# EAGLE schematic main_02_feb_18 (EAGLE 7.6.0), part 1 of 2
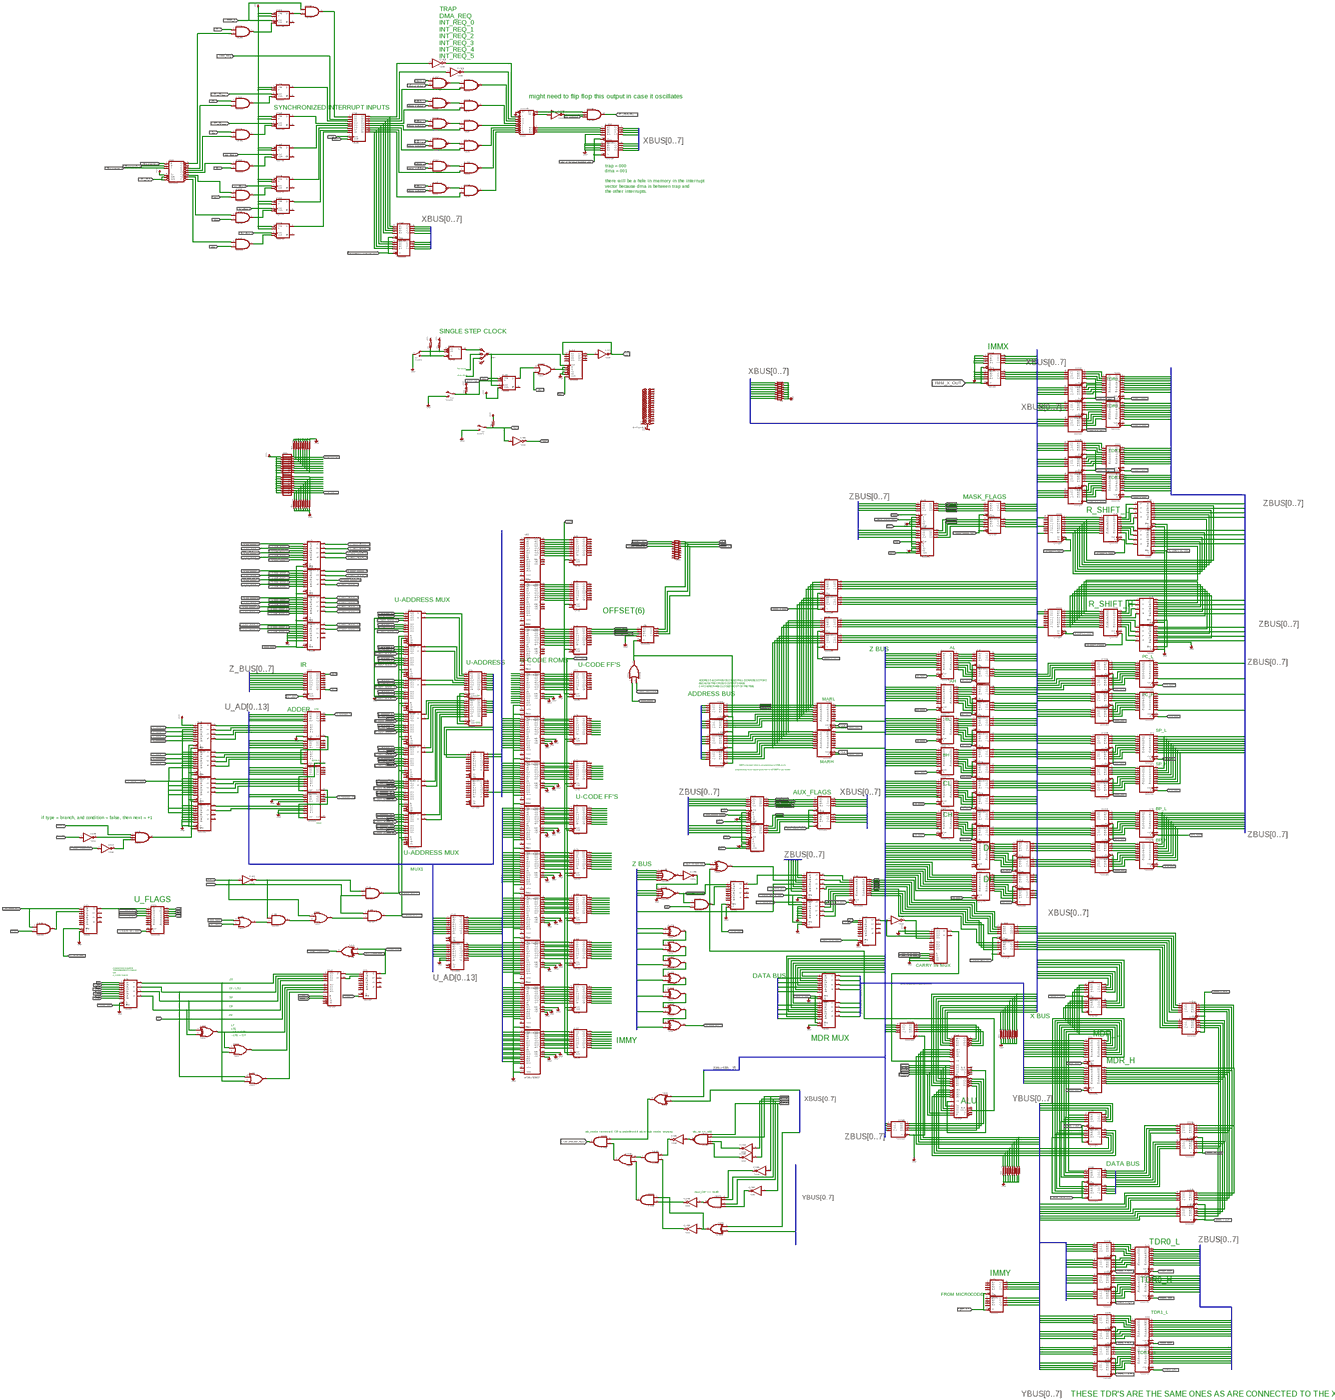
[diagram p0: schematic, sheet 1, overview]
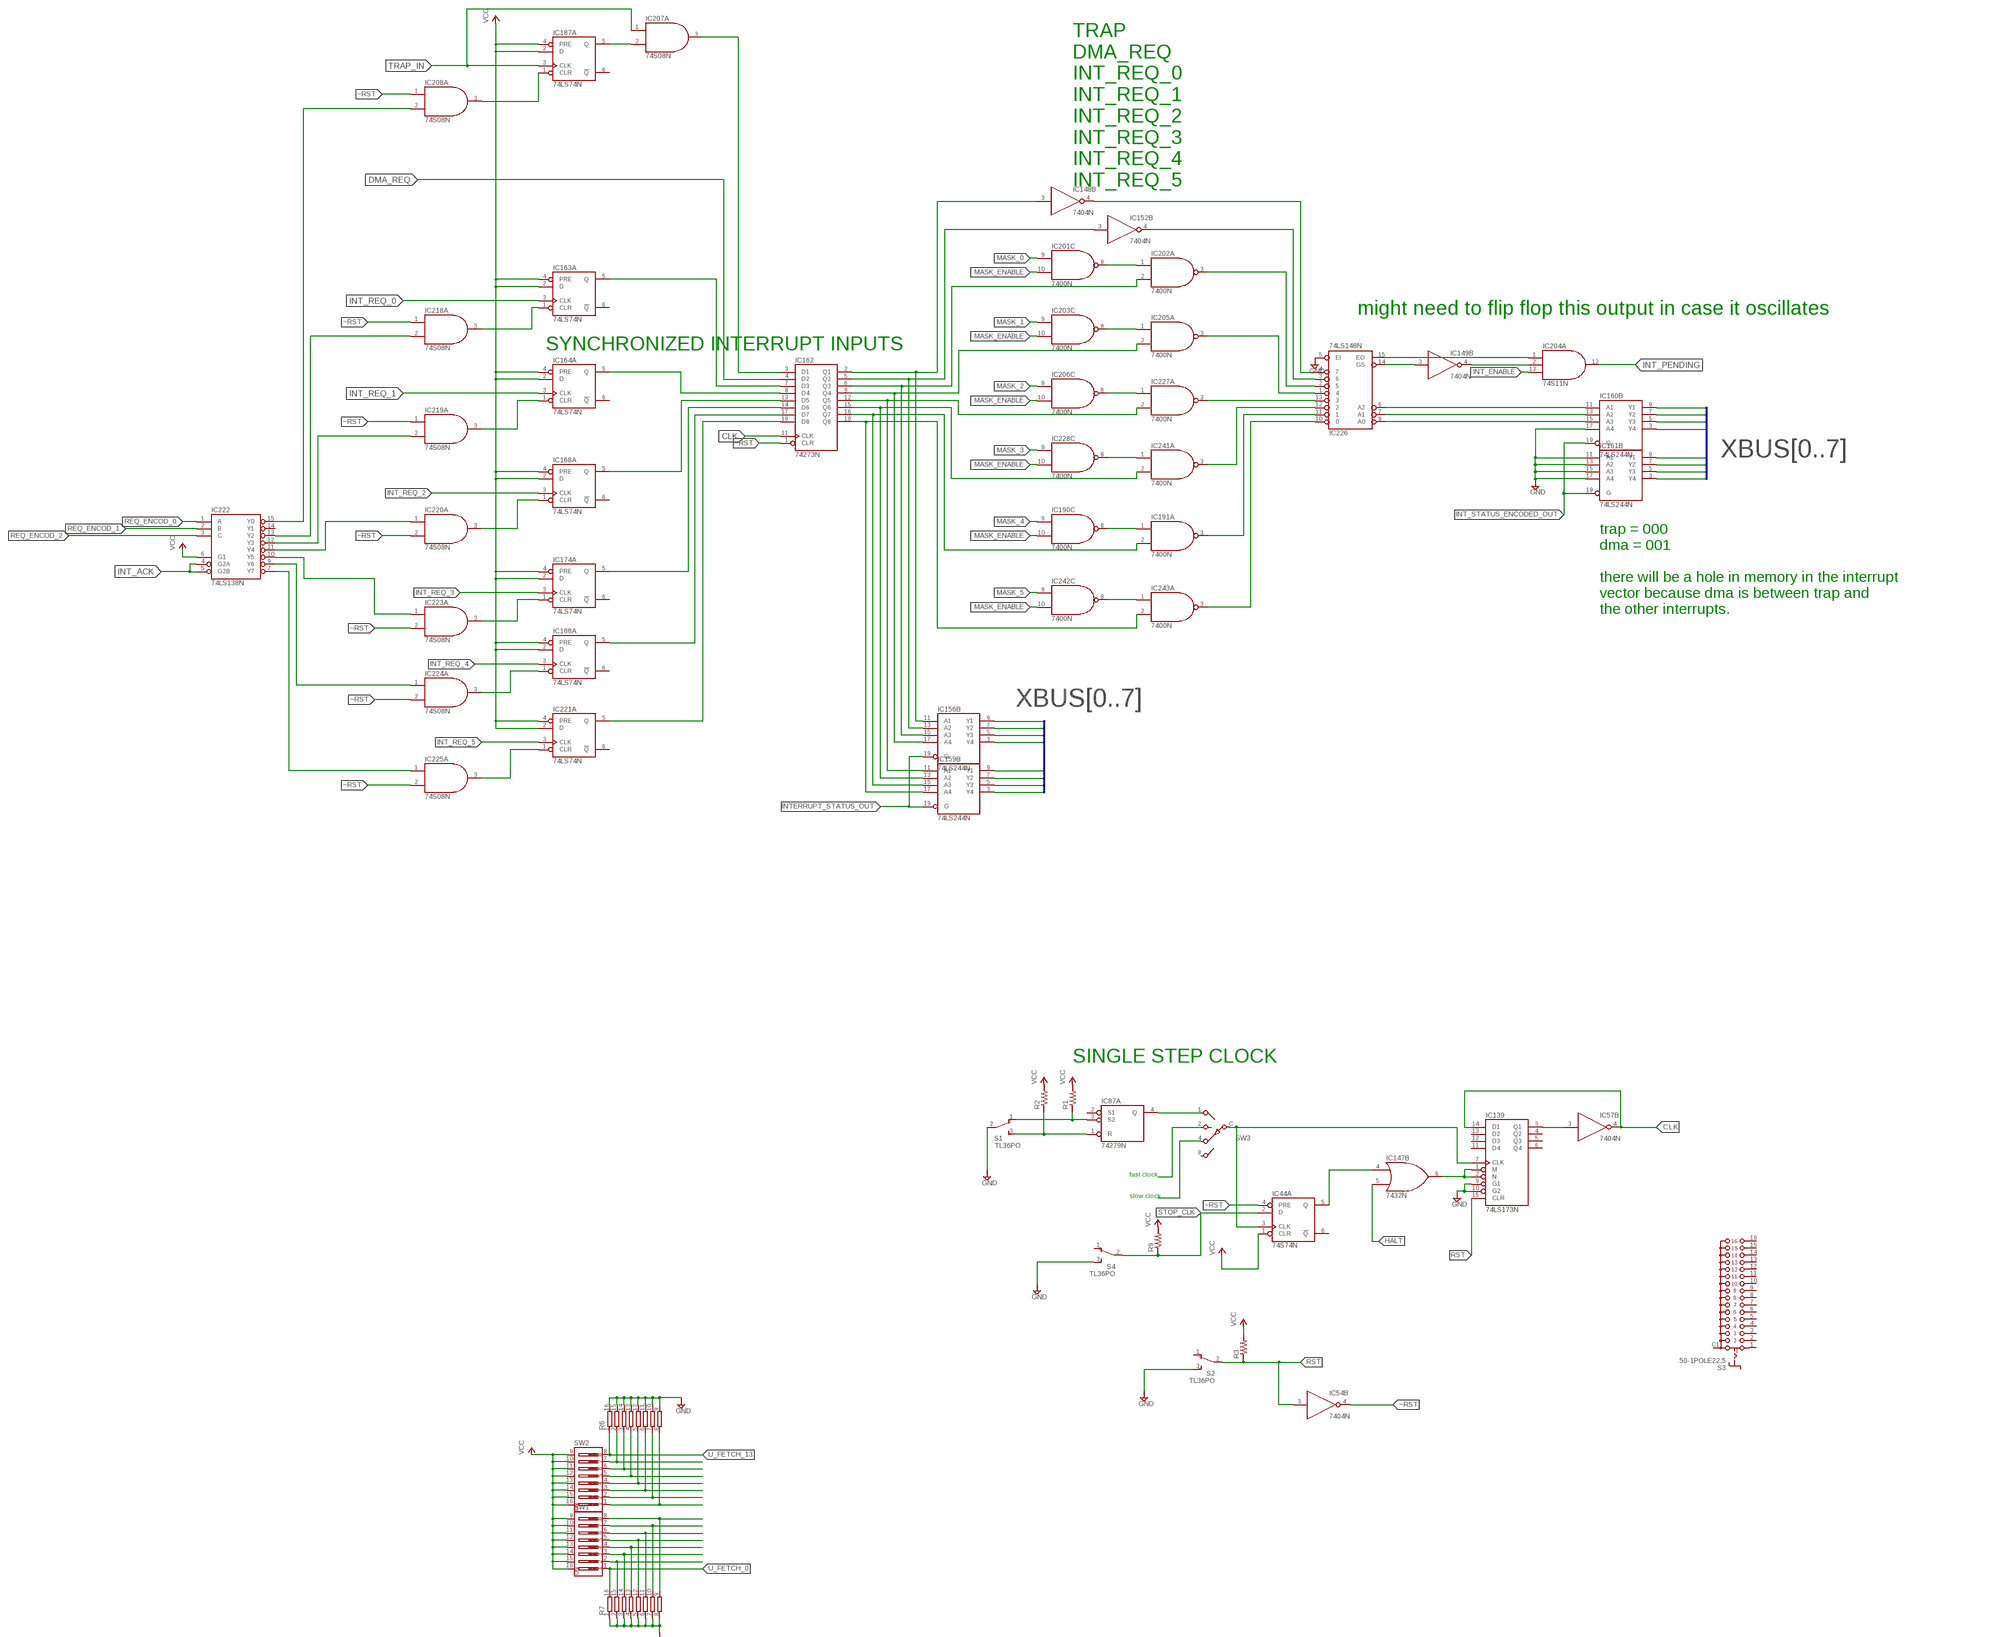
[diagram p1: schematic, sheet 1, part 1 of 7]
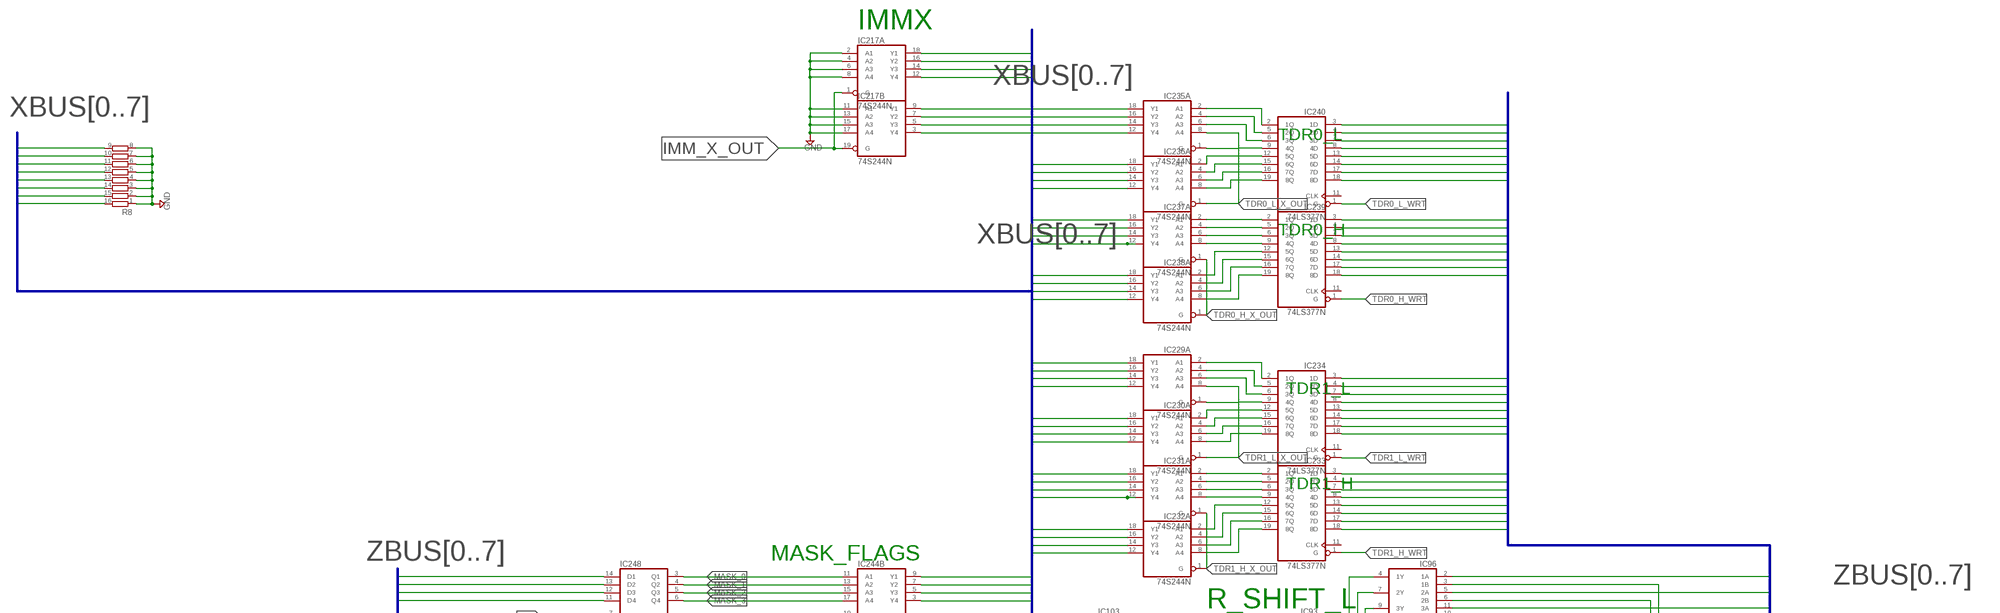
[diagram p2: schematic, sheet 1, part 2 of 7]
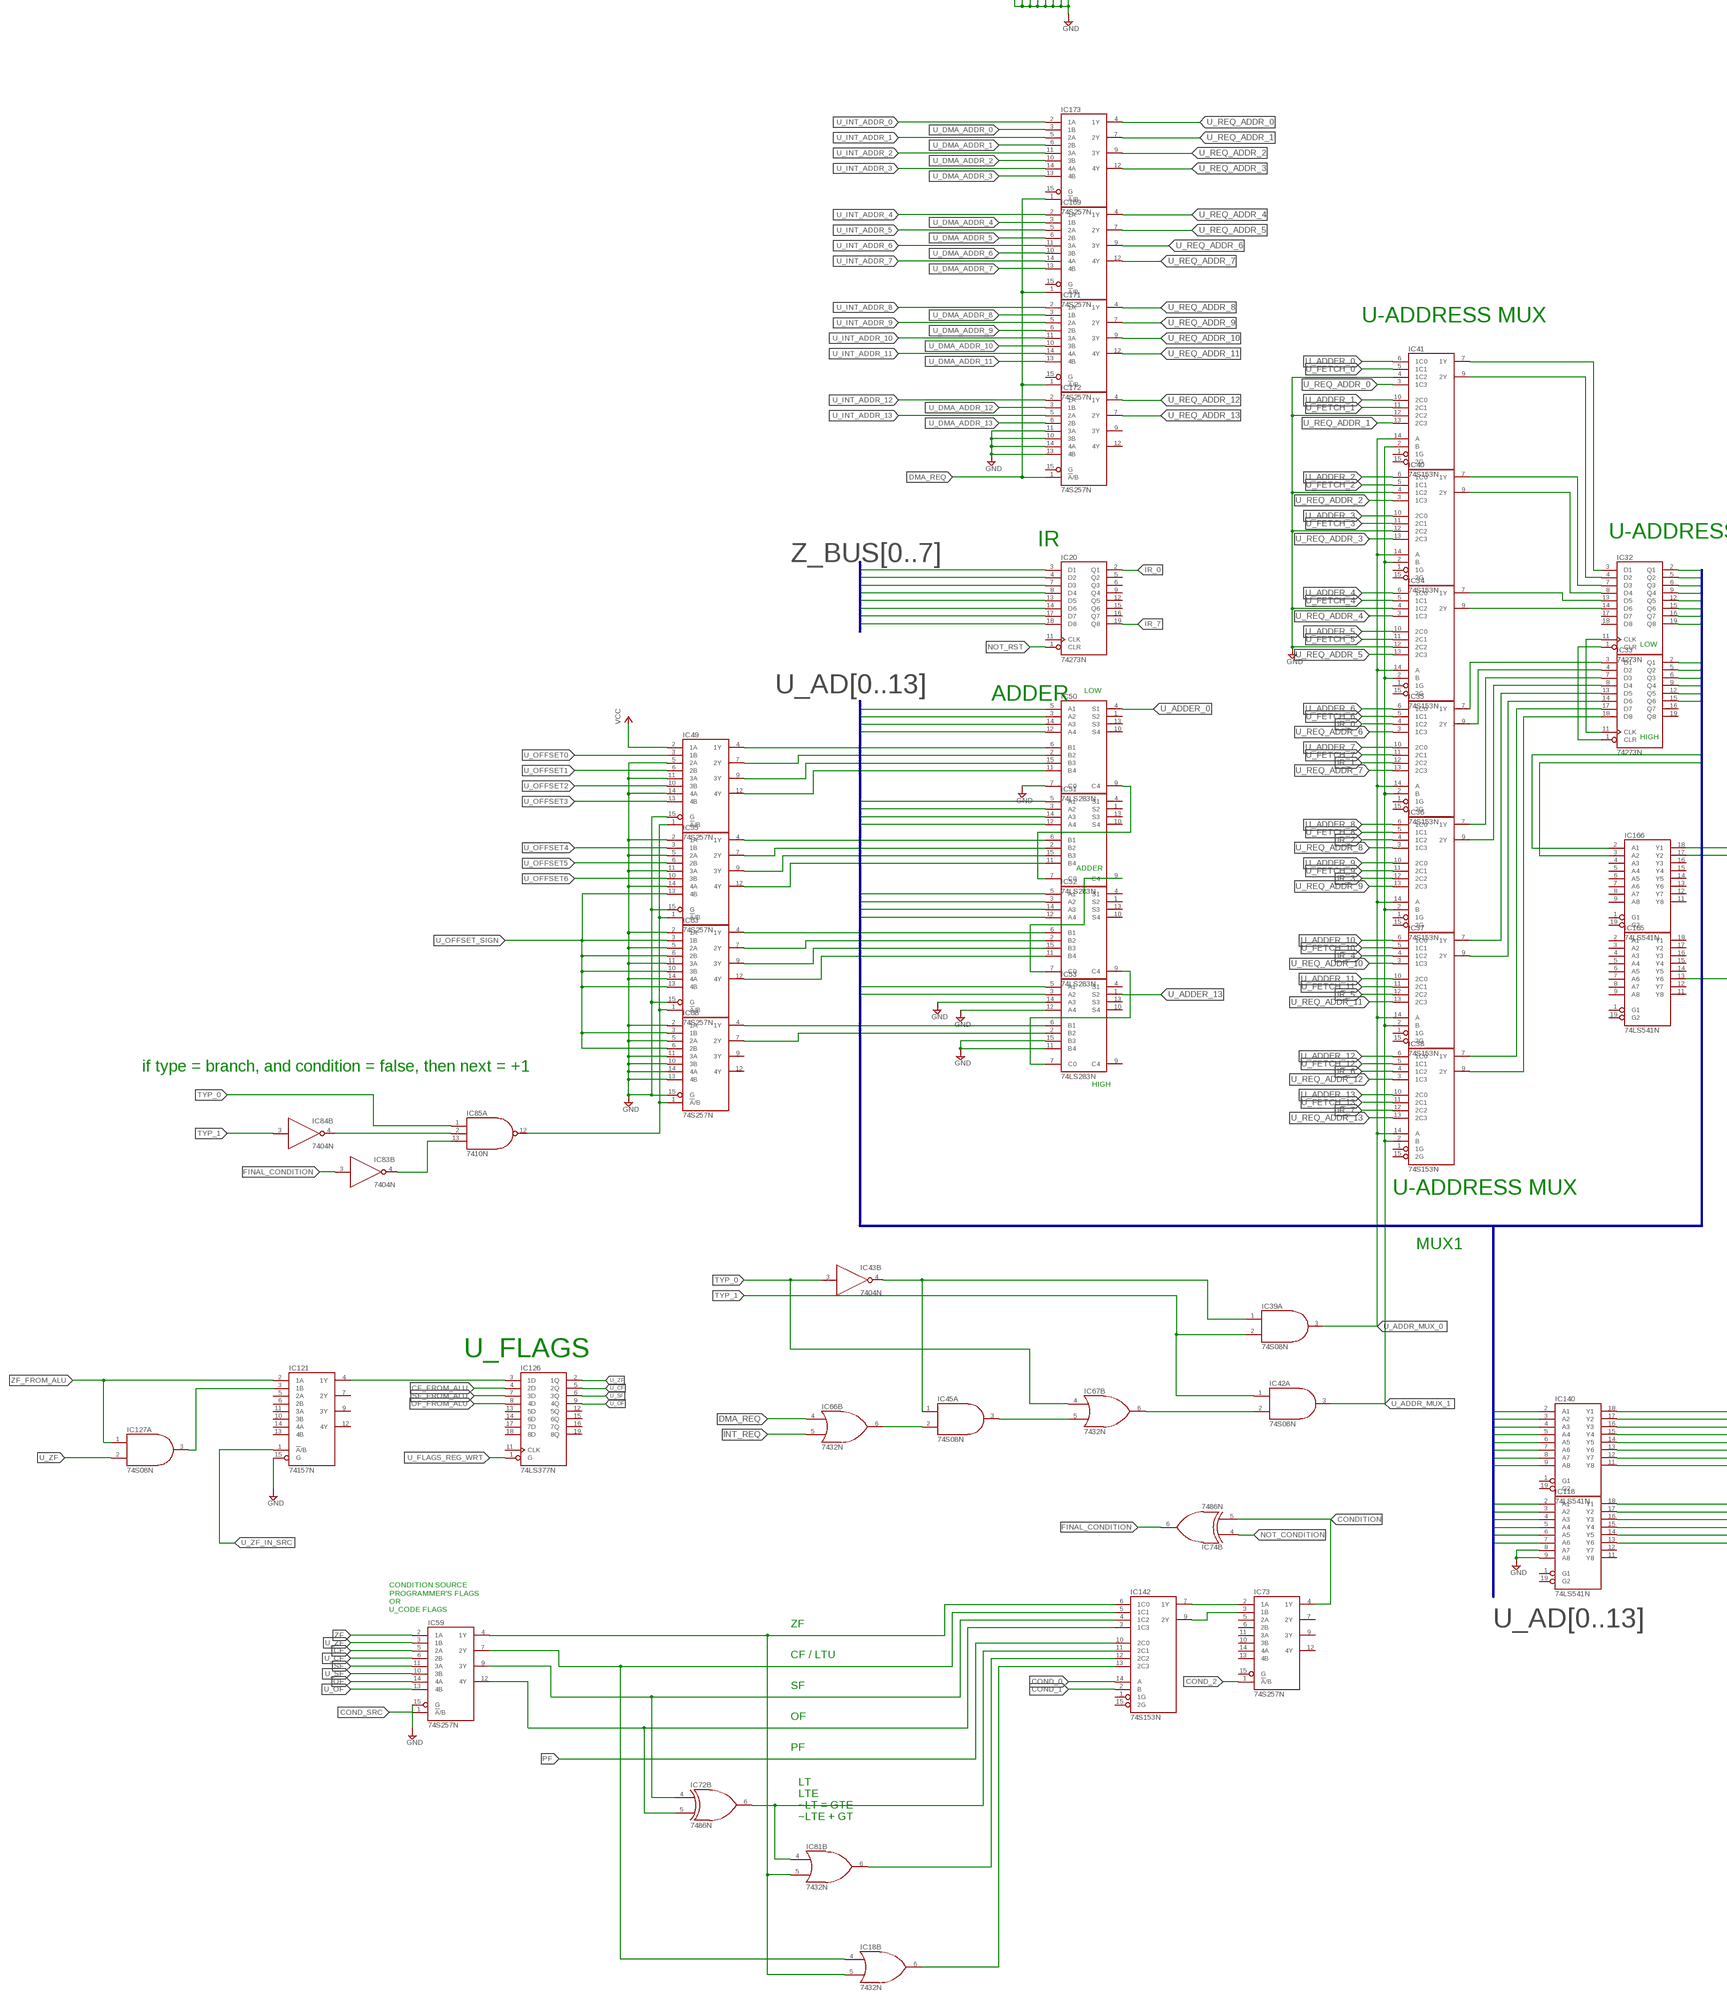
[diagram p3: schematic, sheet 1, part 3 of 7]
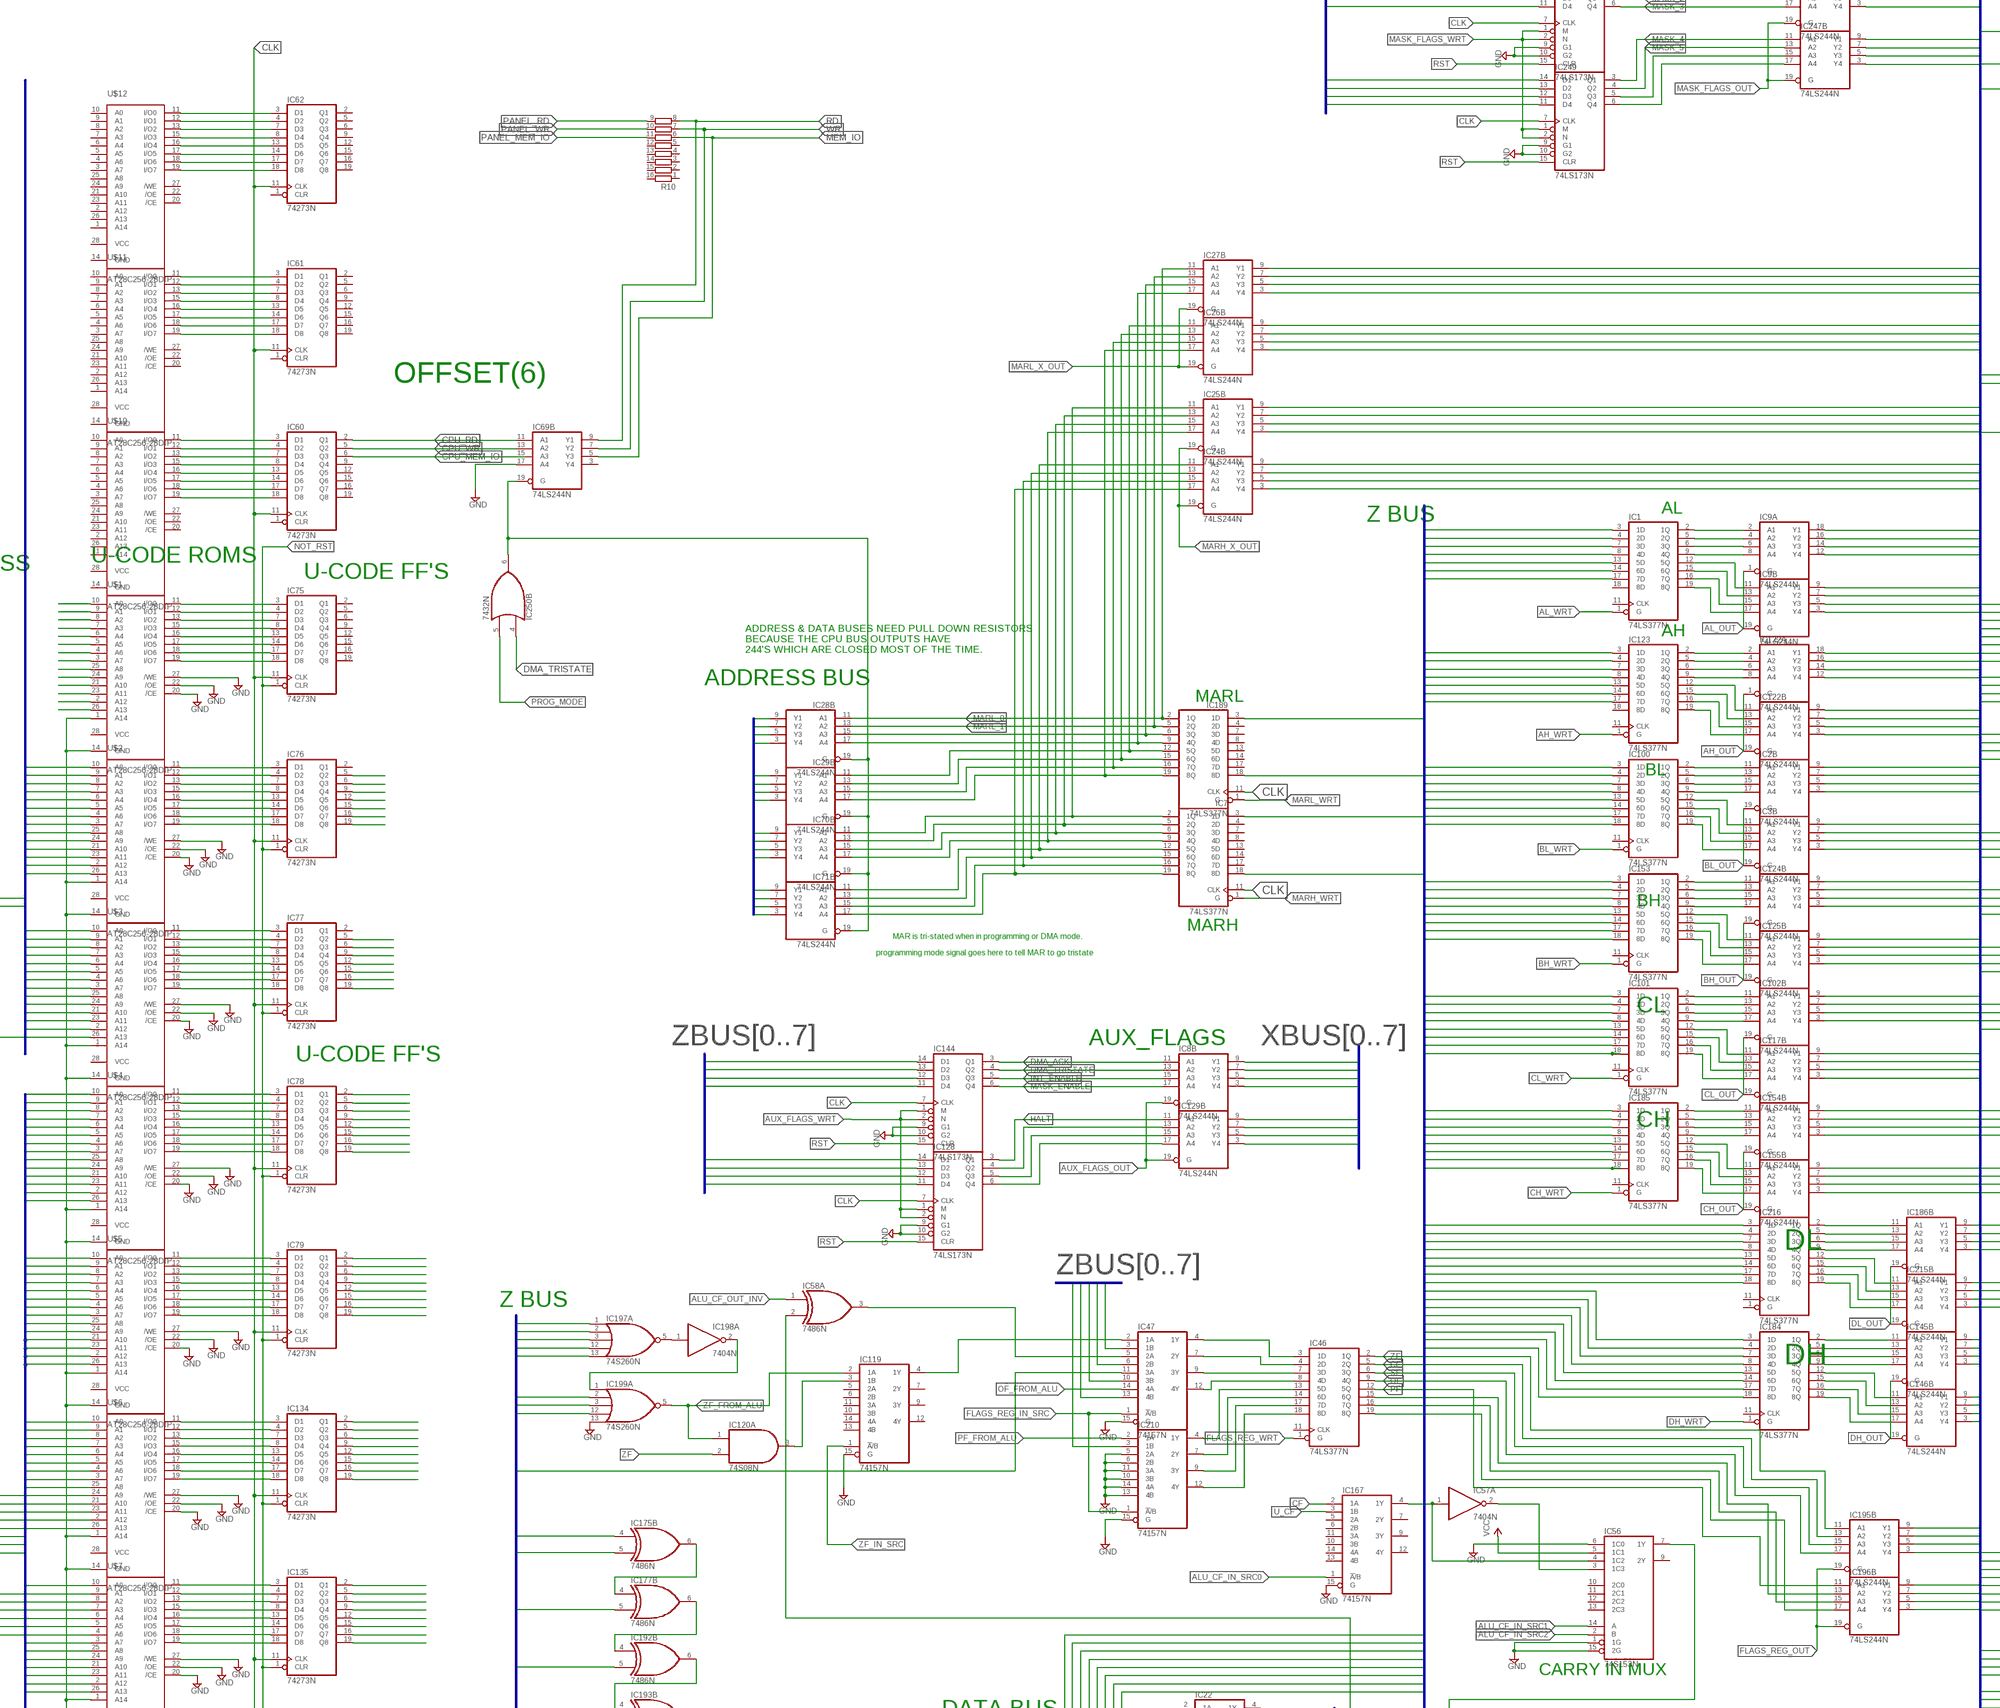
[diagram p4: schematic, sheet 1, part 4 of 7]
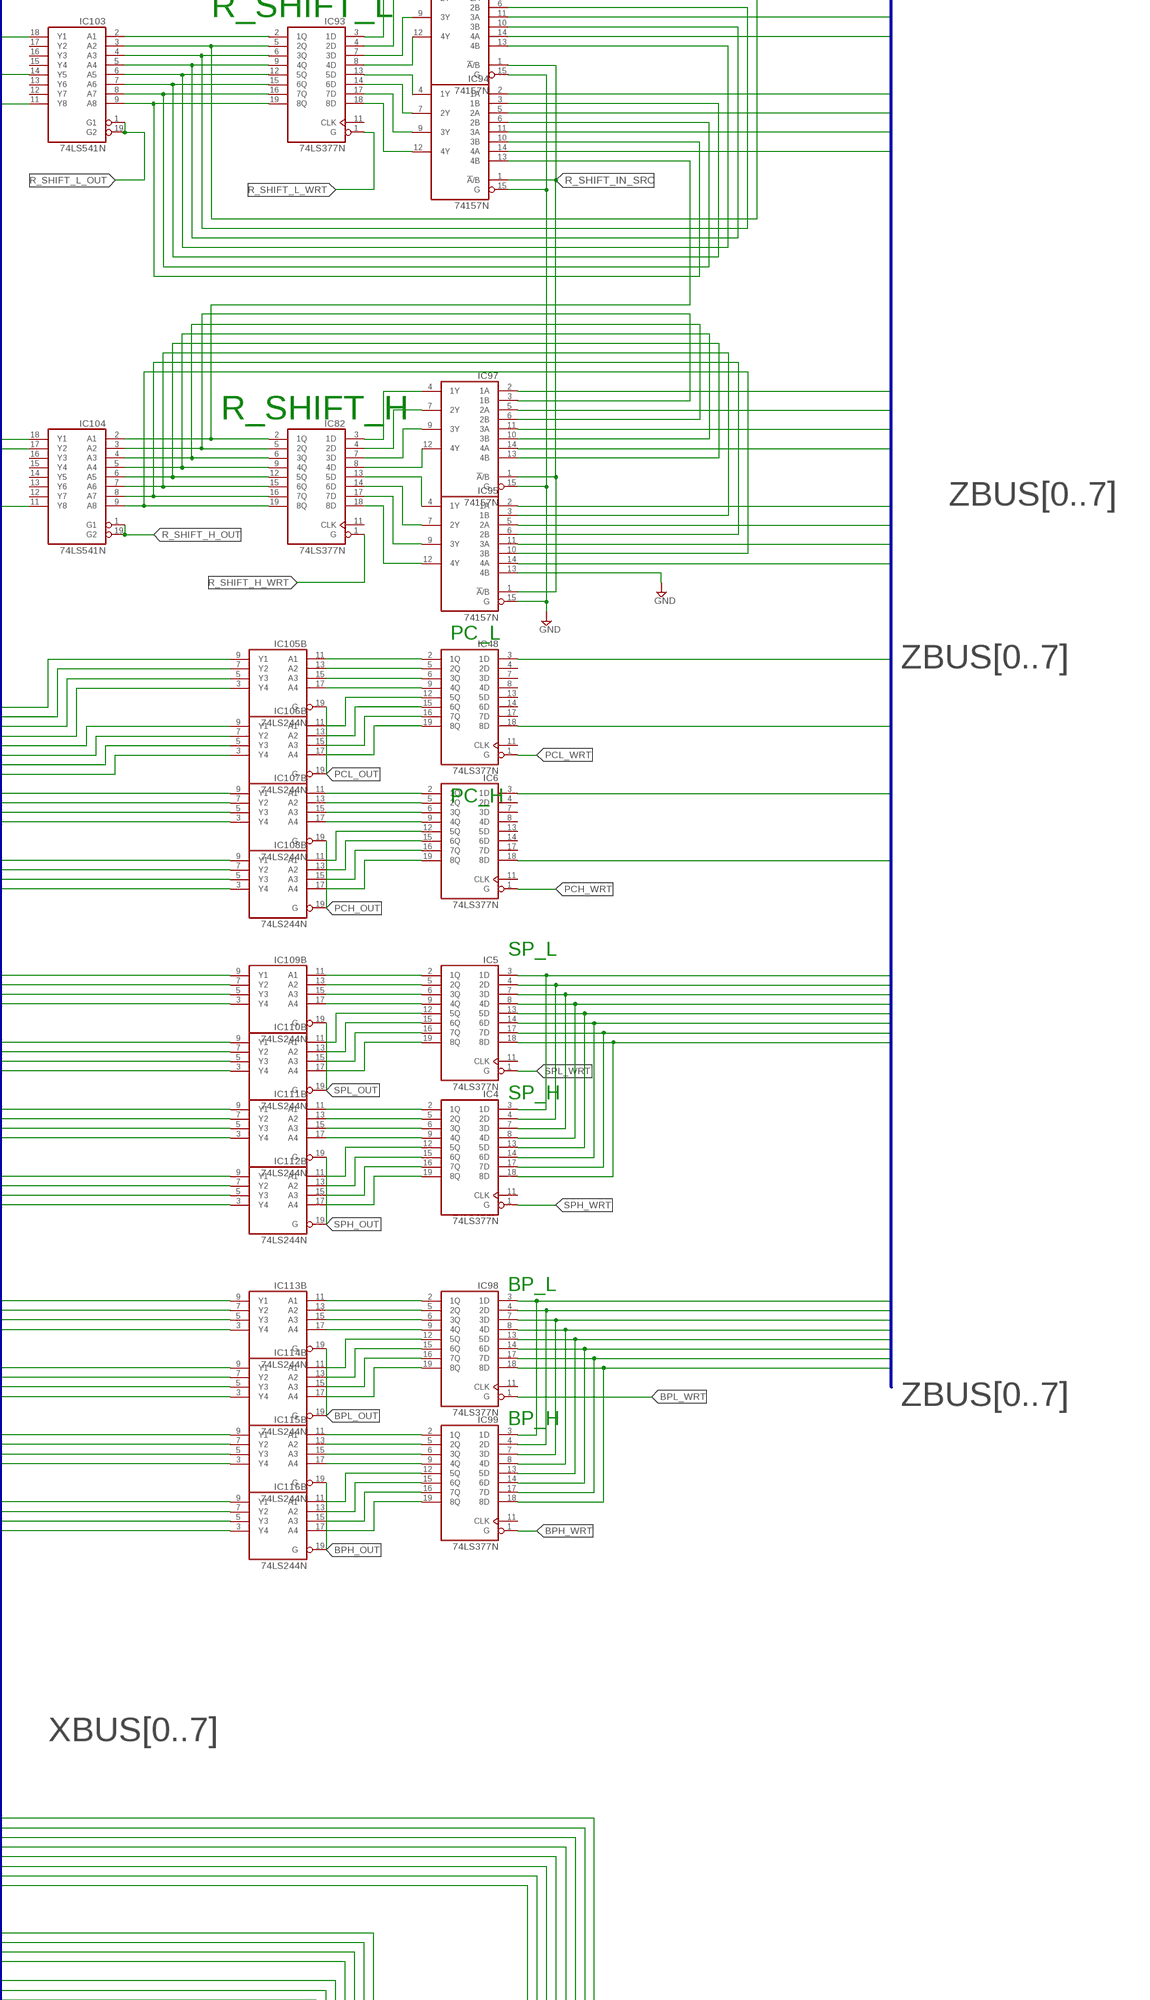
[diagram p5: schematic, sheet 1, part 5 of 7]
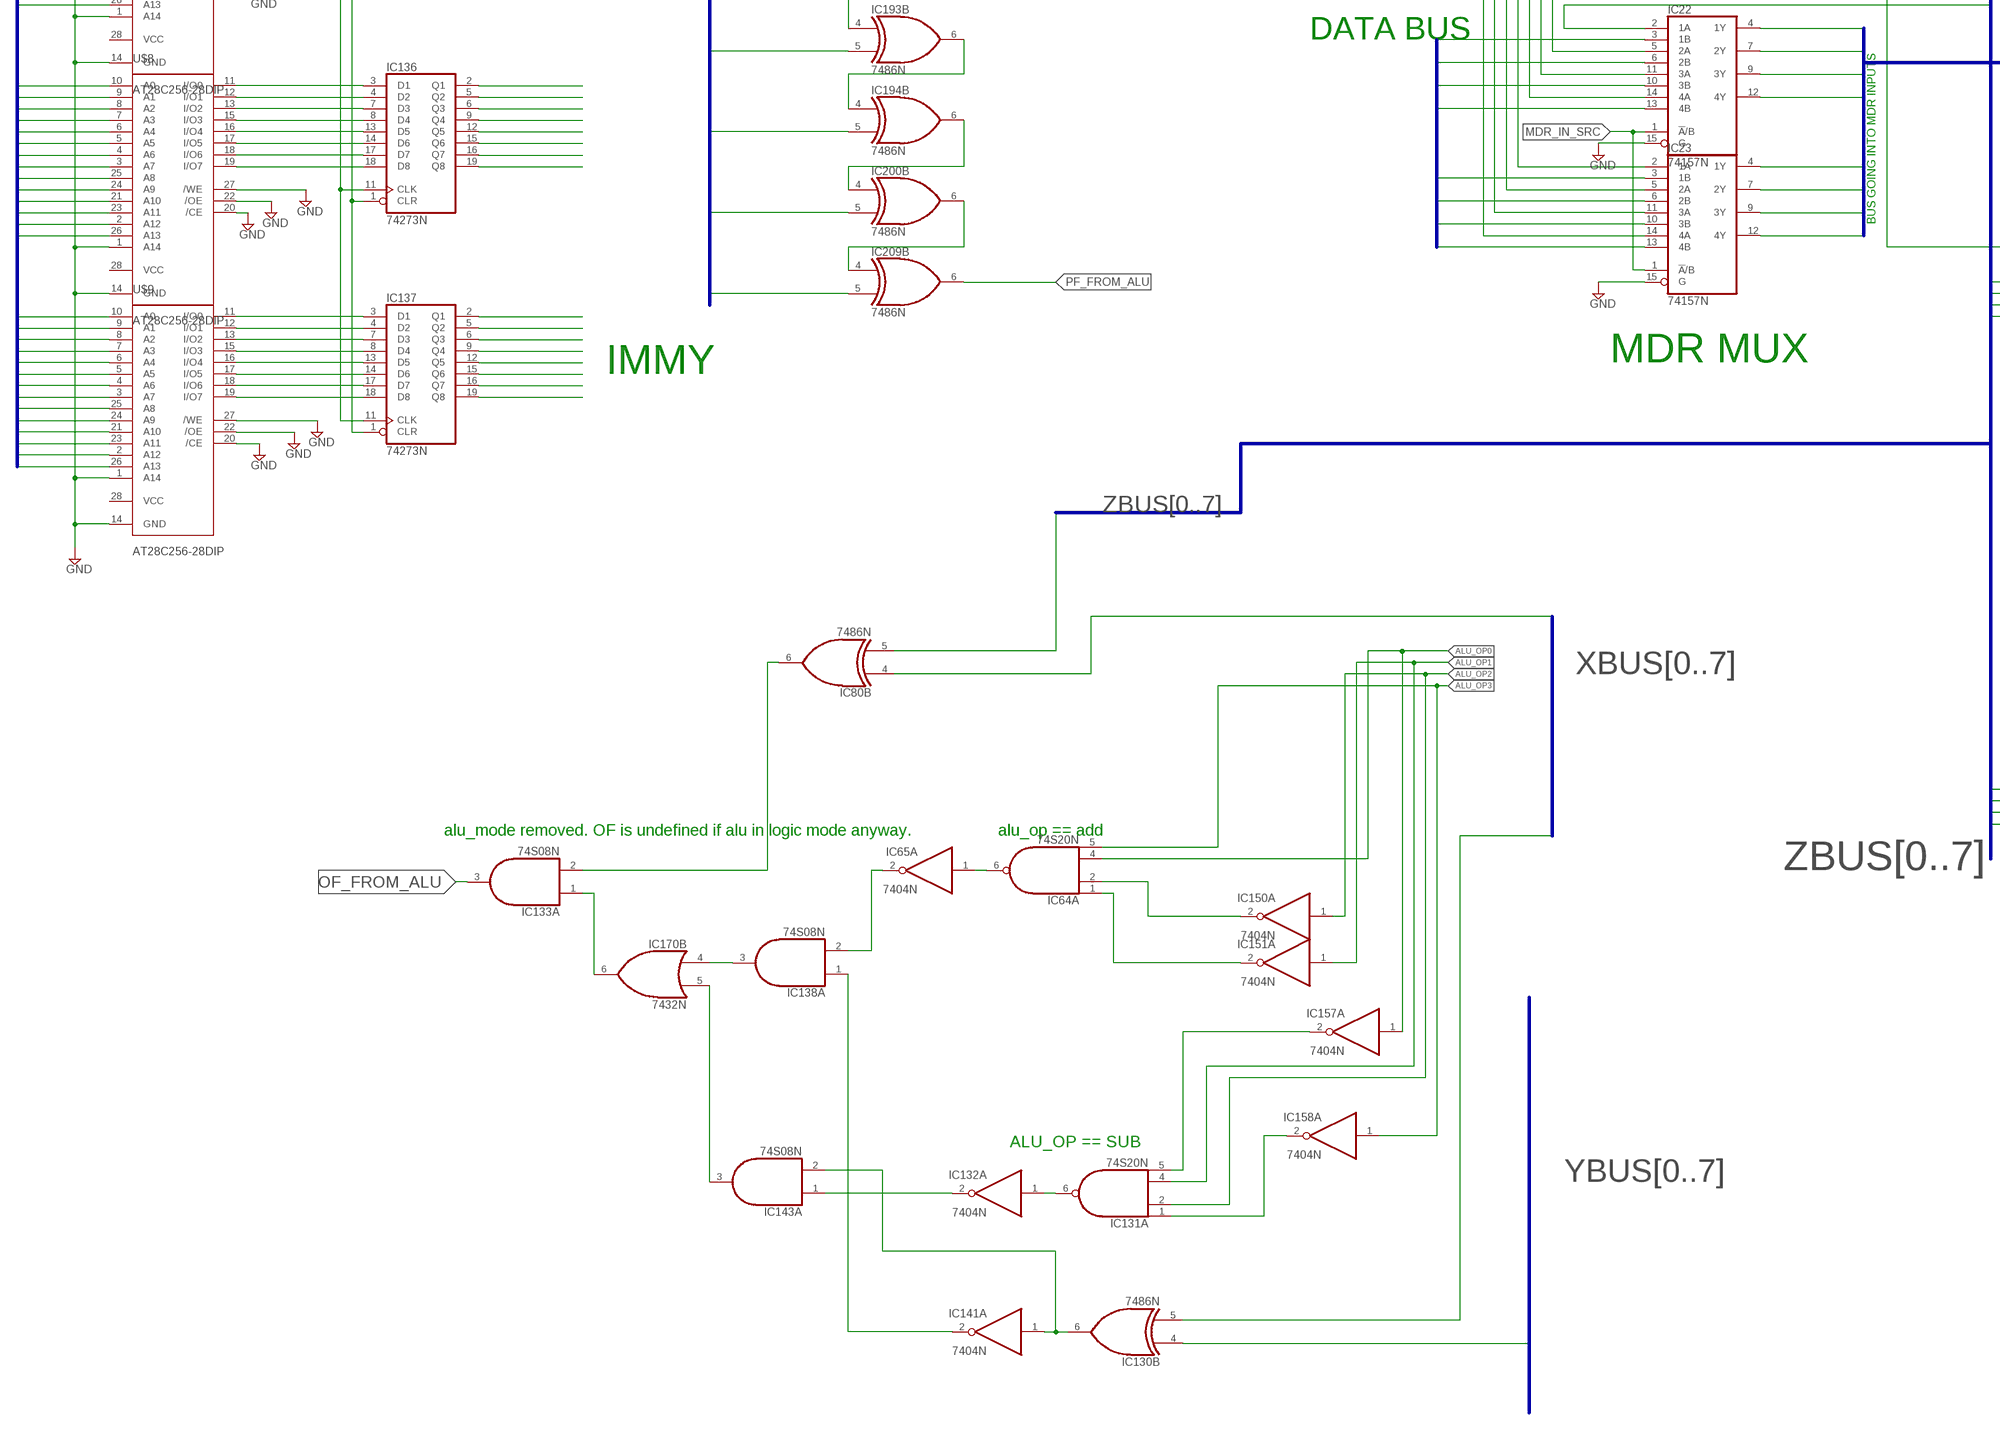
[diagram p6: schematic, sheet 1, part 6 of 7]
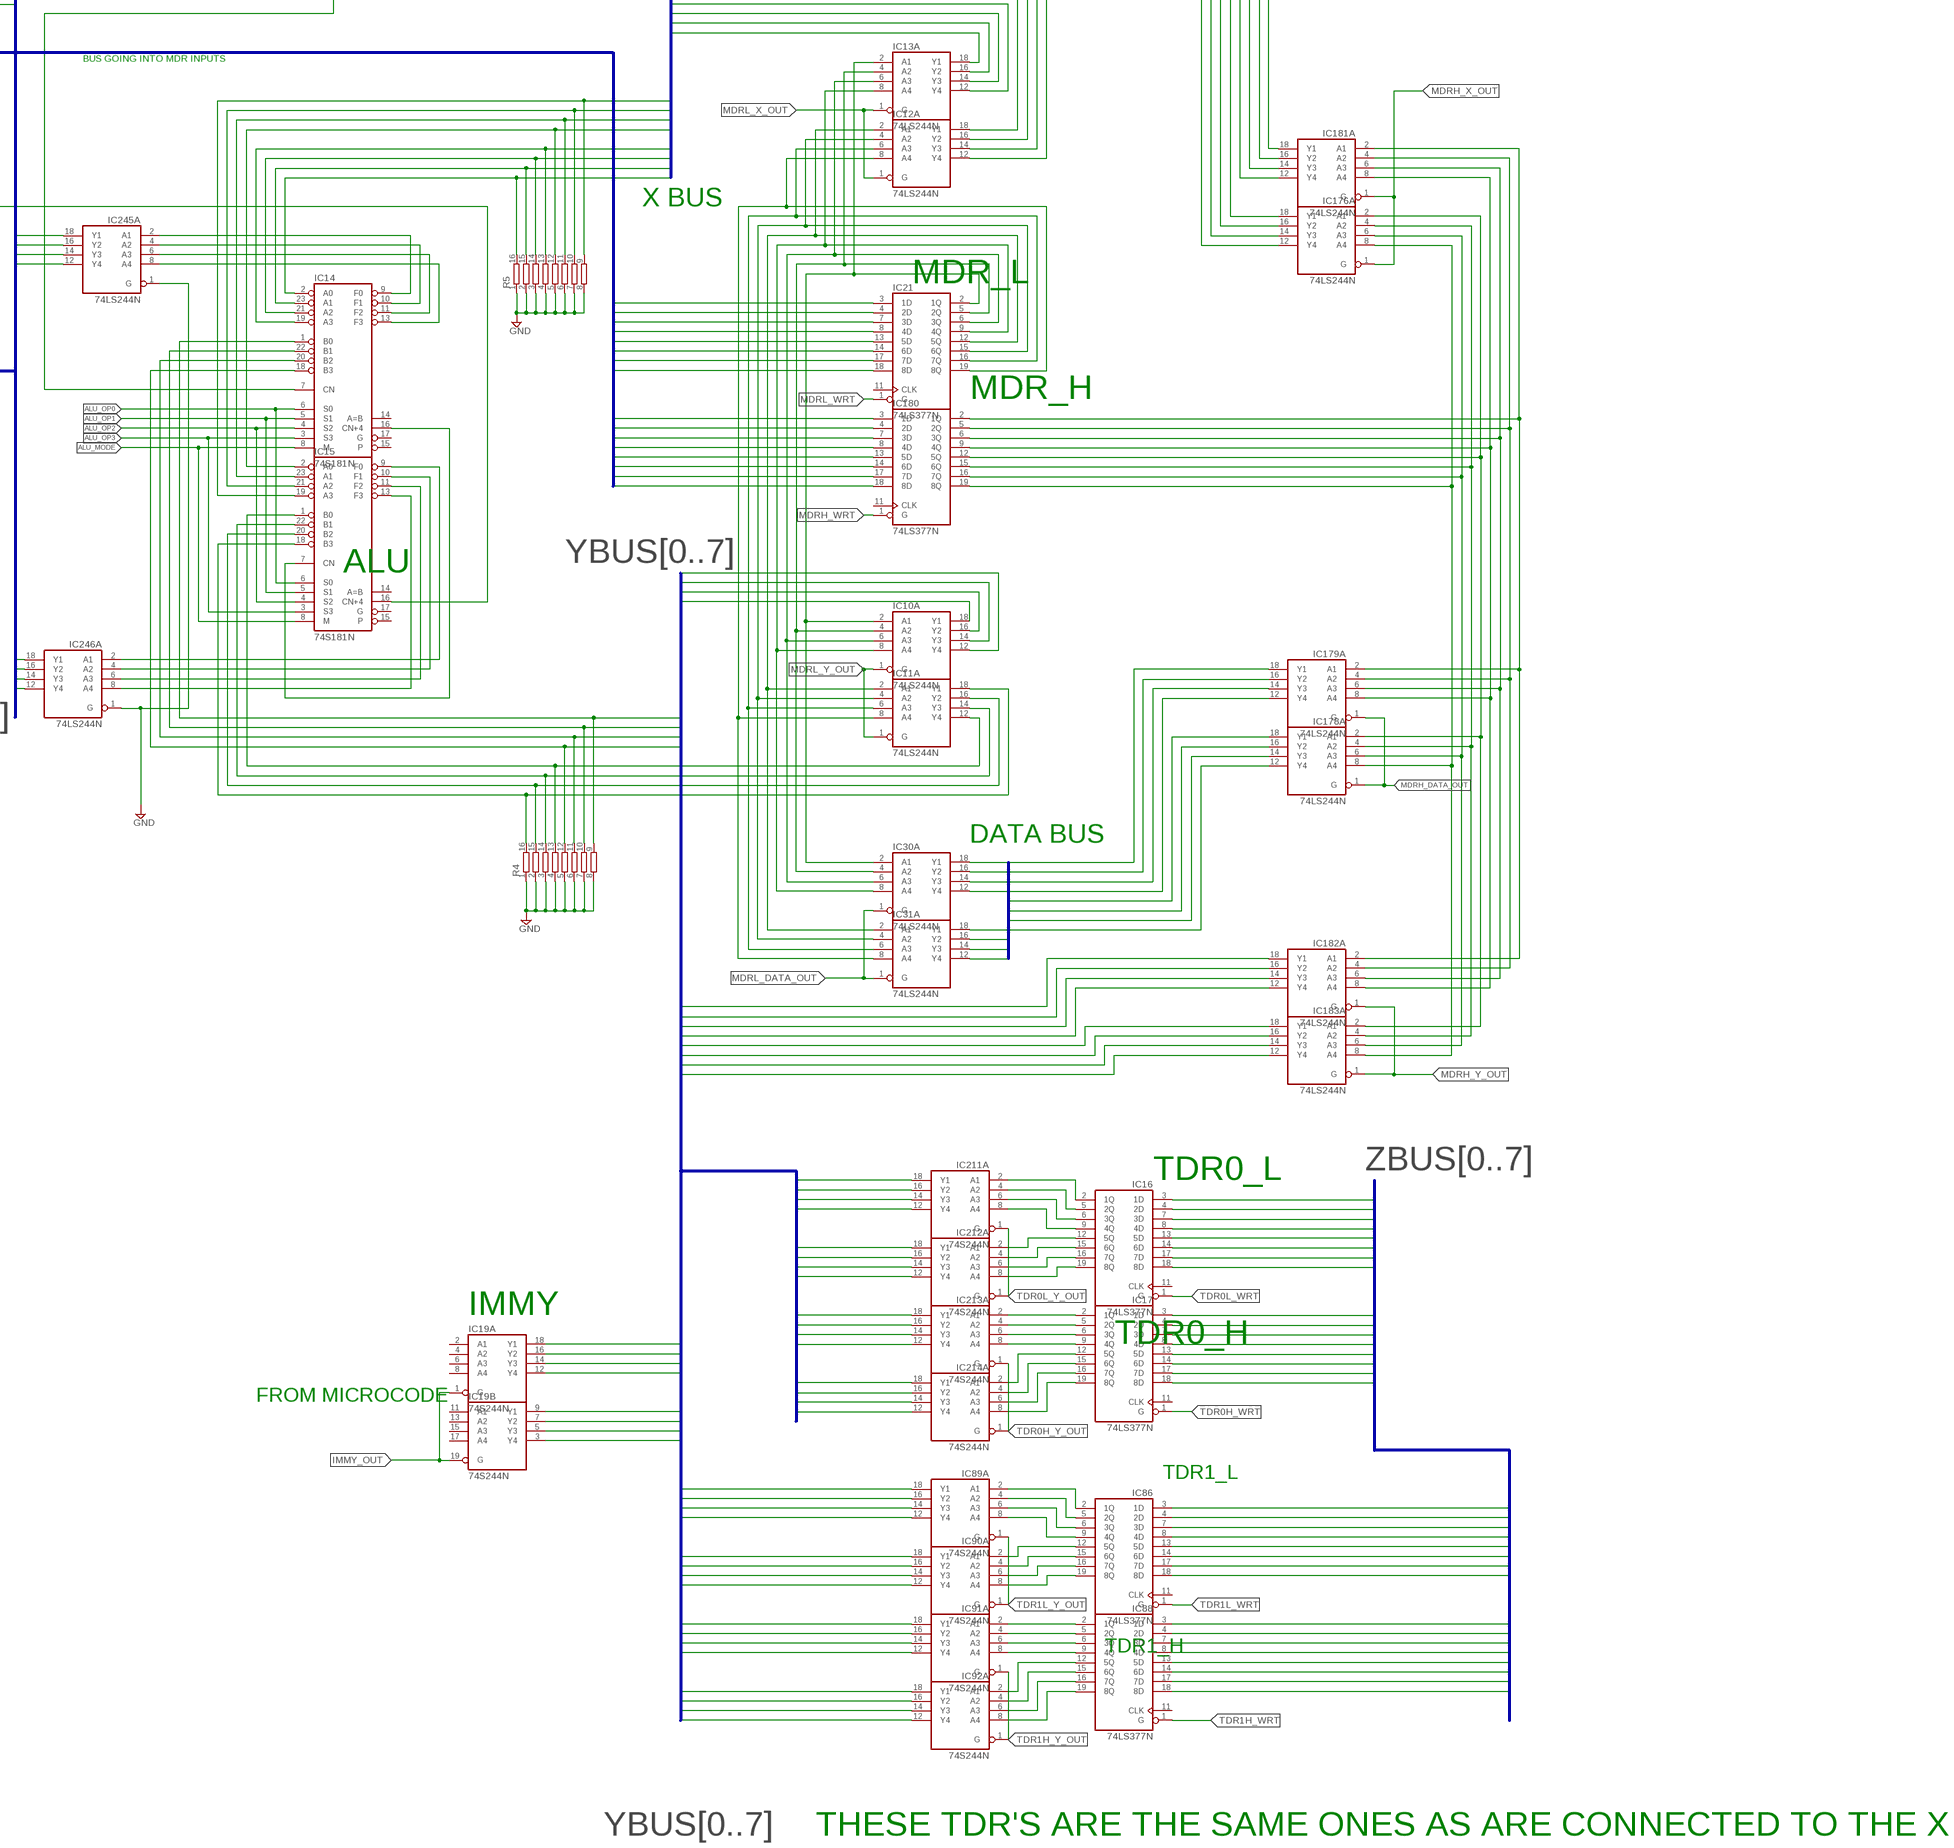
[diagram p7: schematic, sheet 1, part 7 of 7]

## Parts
IC1  74LS377N  [DIL20]
IC2  74LS244N  [DIL20]
IC3  74LS244N  [DIL20]
IC4  74LS377N  [DIL20]
IC5  74LS377N  [DIL20]
IC6  74LS377N  [DIL20]
IC7  74LS377N  [DIL20]
IC8  74LS244N  [DIL20]
IC9  74LS244N  [DIL20]
IC10  74LS244N  [DIL20]
IC11  74LS244N  [DIL20]
IC12  74LS244N  [DIL20]
IC13  74LS244N  [DIL20]
IC14  74S181N  [DIL24-6]
IC15  74S181N  [DIL24-6]
IC16  74LS377N  [DIL20]
IC17  74LS377N  [DIL20]
IC18  7432N  [DIL14]
IC19  74S244N  [DIL20]
IC20  74273N  [DIL20]
IC21  74LS377N  [DIL20]
IC22  74157N  [DIL16]
IC23  74157N  [DIL16]
IC24  74LS244N  [DIL20]
IC25  74LS244N  [DIL20]
IC26  74LS244N  [DIL20]
IC27  74LS244N  [DIL20]
IC28  74LS244N  [DIL20]
IC29  74LS244N  [DIL20]
IC30  74LS244N  [DIL20]
IC31  74LS244N  [DIL20]
IC32  74273N  [DIL20]
IC33  74273N  [DIL20]
IC34  74S153N  [DIL16]
IC35  74S153N  [DIL16]
IC36  74S153N  [DIL16]
IC37  74S153N  [DIL16]
IC38  74S153N  [DIL16]
IC39  74S08N  [DIL14]
IC40  74S153N  [DIL16]
IC41  74S153N  [DIL16]
IC42  74S08N  [DIL14]
IC43  7404N  [DIL14]
IC44  74S74N  [DIL14]
IC45  74S08N  [DIL14]
IC46  74LS377N  [DIL20]
IC47  74157N  [DIL16]
IC48  74LS377N  [DIL20]
IC49  74S257N  [DIL16]
IC50  74LS283N  [DIL16]
IC51  74LS283N  [DIL16]
IC52  74LS283N  [DIL16]
IC53  74LS283N  [DIL16]
IC54  7404N  [DIL14]
IC55  74S257N  [DIL16]
IC56  74S153N  [DIL16]
IC57  7404N  [DIL14]
IC58  7486N  [DIL14]
IC59  74S257N  [DIL16]
IC60  74273N  [DIL20]
IC61  74273N  [DIL20]
IC62  74273N  [DIL20]
IC63  74S257N  [DIL16]
IC64  74S20N  [DIL14]
IC65  7404N  [DIL14]
IC66  7432N  [DIL14]
IC67  7432N  [DIL14]
IC68  74S257N  [DIL16]
IC69  74LS244N  [DIL20]
IC70  74LS244N  [DIL20]
IC71  74LS244N  [DIL20]
IC72  7486N  [DIL14]
IC73  74S257N  [DIL16]
IC74  7486N  [DIL14]
IC75  74273N  [DIL20]
IC76  74273N  [DIL20]
IC77  74273N  [DIL20]
IC78  74273N  [DIL20]
IC79  74273N  [DIL20]
IC80  7486N  [DIL14]
IC81  7432N  [DIL14]
IC82  74LS377N  [DIL20]
IC83  7404N  [DIL14]
IC84  7404N  [DIL14]
IC85  7410N  [DIL14]
IC86  74LS377N  [DIL20]
IC87  74279N  [DIL16]
IC88  74LS377N  [DIL20]
IC89  74S244N  [DIL20]
IC90  74S244N  [DIL20]
IC91  74S244N  [DIL20]
IC92  74S244N  [DIL20]
IC93  74LS377N  [DIL20]
IC94  74157N  [DIL16]
IC95  74157N  [DIL16]
IC96  74157N  [DIL16]
IC97  74157N  [DIL16]
IC98  74LS377N  [DIL20]
IC99  74LS377N  [DIL20]
IC100  74LS377N  [DIL20]
IC101  74LS377N  [DIL20]
IC102  74LS244N  [DIL20]
IC103  74LS541N  [DIL20]
IC104  74LS541N  [DIL20]
IC105  74LS244N  [DIL20]
IC106  74LS244N  [DIL20]
IC107  74LS244N  [DIL20]
IC108  74LS244N  [DIL20]
IC109  74LS244N  [DIL20]
IC110  74LS244N  [DIL20]
IC111  74LS244N  [DIL20]
IC112  74LS244N  [DIL20]
IC113  74LS244N  [DIL20]
IC114  74LS244N  [DIL20]
IC115  74LS244N  [DIL20]
IC116  74LS244N  [DIL20]
IC117  74LS244N  [DIL20]
IC118  74LS541N  [DIL20]
IC119  74157N  [DIL16]
IC120  74S08N  [DIL14]
IC121  74157N  [DIL16]
IC122  74LS244N  [DIL20]
IC123  74LS377N  [DIL20]
IC124  74LS244N  [DIL20]
IC125  74LS244N  [DIL20]
IC126  74LS377N  [DIL20]
IC127  74S08N  [DIL14]
IC128  74LS173N  [DIL16]
IC129  74LS244N  [DIL20]
IC130  7486N  [DIL14]
IC131  74S20N  [DIL14]
IC132  7404N  [DIL14]
IC133  74S08N  [DIL14]
IC134  74273N  [DIL20]
IC135  74273N  [DIL20]
IC136  74273N  [DIL20]
IC137  74273N  [DIL20]
IC138  74S08N  [DIL14]
IC139  74LS173N  [DIL16]
IC140  74LS541N  [DIL20]
IC141  7404N  [DIL14]
IC142  74S153N  [DIL16]
IC143  74S08N  [DIL14]
IC144  74LS173N  [DIL16]
IC145  74LS244N  [DIL20]
IC146  74LS244N  [DIL20]
IC147  7432N  [DIL14]
IC148  7404N  [DIL14]
IC149  7404N  [DIL14]
IC150  7404N  [DIL14]
IC151  7404N  [DIL14]
IC152  7404N  [DIL14]
IC153  74LS377N  [DIL20]
IC154  74LS244N  [DIL20]
IC155  74LS244N  [DIL20]
IC156  74LS244N  [DIL20]
IC157  7404N  [DIL14]
IC158  7404N  [DIL14]
IC159  74LS244N  [DIL20]
IC160  74LS244N  [DIL20]
IC161  74LS244N  [DIL20]
IC162  74273N  [DIL20]
IC163  74LS74N  [DIL14]
IC164  74LS74N  [DIL14]
IC165  74LS541N  [DIL20]
IC166  74LS541N  [DIL20]
IC167  74157N  [DIL16]
IC168  74LS74N  [DIL14]
IC169  74S257N  [DIL16]
IC170  7432N  [DIL14]
IC171  74S257N  [DIL16]
IC172  74S257N  [DIL16]
IC173  74S257N  [DIL16]
IC174  74LS74N  [DIL14]
IC175  7486N  [DIL14]
IC176  74LS244N  [DIL20]
IC177  7486N  [DIL14]
IC178  74LS244N  [DIL20]
IC179  74LS244N  [DIL20]
IC180  74LS377N  [DIL20]
IC181  74LS244N  [DIL20]
IC182  74LS244N  [DIL20]
IC183  74LS244N  [DIL20]
IC184  74LS377N  [DIL20]
IC185  74LS377N  [DIL20]
IC186  74LS244N  [DIL20]
IC187  74LS74N  [DIL14]
IC188  74LS74N  [DIL14]
IC189  74LS377N  [DIL20]
IC190  7400N  [DIL14]
IC191  7400N  [DIL14]
IC192  7486N  [DIL14]
IC193  7486N  [DIL14]
IC194  7486N  [DIL14]
IC195  74LS244N  [DIL20]
IC196  74LS244N  [DIL20]
IC197  74S260N  [DIL14]
IC198  7404N  [DIL14]
IC199  74S260N  [DIL14]
IC200  7486N  [DIL14]
IC201  7400N  [DIL14]
IC202  7400N  [DIL14]
IC203  7400N  [DIL14]
IC204  74S11N  [DIL14]
IC205  7400N  [DIL14]
IC206  7400N  [DIL14]
IC207  74S08N  [DIL14]
IC208  74S08N  [DIL14]
IC209  7486N  [DIL14]
IC210  74157N  [DIL16]
IC211  74S244N  [DIL20]
IC212  74S244N  [DIL20]
IC213  74S244N  [DIL20]
IC214  74S244N  [DIL20]
IC215  74LS244N  [DIL20]
IC216  74LS377N  [DIL20]
IC217  74S244N  [DIL20]
IC218  74S08N  [DIL14]
IC219  74S08N  [DIL14]
IC220  74S08N  [DIL14]
IC221  74LS74N  [DIL14]
IC222  74LS138N  [DIL16]
IC223  74S08N  [DIL14]
IC224  74S08N  [DIL14]
IC225  74S08N  [DIL14]
IC226  74LS148N  [DIL16]
IC227  7400N  [DIL14]
IC228  7400N  [DIL14]
IC229  74S244N  [DIL20]
IC230  74S244N  [DIL20]
IC231  74S244N  [DIL20]
IC232  74S244N  [DIL20]
IC233  74LS377N  [DIL20]
IC234  74LS377N  [DIL20]
IC235  74S244N  [DIL20]
IC236  74S244N  [DIL20]
IC237  74S244N  [DIL20]
IC238  74S244N  [DIL20]
IC239  74LS377N  [DIL20]
IC240  74LS377N  [DIL20]
IC241  7400N  [DIL14]
IC242  7400N  [DIL14]
IC243  7400N  [DIL14]
IC244  74LS244N  [DIL20]
IC245  74LS244N  [DIL20]
IC246  74LS244N  [DIL20]
IC247  74LS244N  [DIL20]
IC248  74LS173N  [DIL16]
IC249  74LS173N  [DIL16]
IC250  7432N  [DIL14]
R1  R-US_0204/2V  [0204V]
R2  R-US_0204/2V  [0204V]
R3  R-US_0204/2V  [0204V]
R4  4816P-T01  [4816P]
R5  4816P-T01  [4816P]
R6  4816P-T01  [4816P]
R7  4816P-T01  [4816P]
R8  4816P-T01  [4816P]
R9  R-US_0204/2V  [0204V]
R10  4816P-T01  [4816P]
S1  TL36PO  [TL3XPO]
S2  TL36PO  [TL3XPO]
S3  50-1POLE22,5  [50-1POLE22,5]
S4  TL36PO  [TL3XPO]
SW1  SW_DIP-8  [EDG-08]
SW2  SW_DIP-8  [EDG-08]
SW3  SW-C10  [SW-C10]
U$1  AT28C256-28DIP  [DIL28-6]
U$2  AT28C256-28DIP  [DIL28-6]
U$3  AT28C256-28DIP  [DIL28-6]
U$4  AT28C256-28DIP  [DIL28-6]
U$5  AT28C256-28DIP  [DIL28-6]
U$6  AT28C256-28DIP  [DIL28-6]
U$7  AT28C256-28DIP  [DIL28-6]
U$8  AT28C256-28DIP  [DIL28-6]
U$9  AT28C256-28DIP  [DIL28-6]
U$10  AT28C256-28DIP  [DIL28-6]
U$11  AT28C256-28DIP  [DIL28-6]
U$12  AT28C256-28DIP  [DIL28-6]

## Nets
45435: IC18.5(B:I1) IC59.4(1Y) IC81.5(B:I1) IC142.6(1C0)
345345: IC59.9(3Y) IC72.4(B:I0) IC142.4(1C2)
634354: IC18.4(B:I0) IC59.7(2Y) IC142.5(1C1)
654654: IC46.16(7Q) IC196.15(B:A3)
4654654: IC59.12(4Y) IC72.5(B:I1) IC142.3(1C3)
5434534: IC46.15(6Q) IC196.13(B:A2)
AD0: IC28.9(B:Y1)
AD1: IC28.7(B:Y2)
AD2: IC28.5(B:Y3)
AD3: IC28.3(B:Y4)
AD4: IC29.9(B:Y1)
AD5: IC29.7(B:Y2)
AD6: IC29.5(B:Y3)
AD7: IC29.3(B:Y4)
AD8: IC70.9(B:Y1)
AD9: IC70.7(B:Y2)
AD10: IC70.5(B:Y3)
AD11: IC70.3(B:Y4)
AD12: IC71.9(B:Y1)
AD13: IC71.7(B:Y2)
AD14: IC71.5(B:Y3)
AD15: IC71.3(B:Y4)
AH_OUT: IC122.1(A:G) IC122.19(B:G)
AH_WRT: IC123.1(G)
AL_OUT: IC9.1(A:G) IC9.19(B:G)
AL_WRT: IC1.1(G)
ALU_CF_IN_SRC0: IC167.1(!A!/B)
ALU_CF_IN_SRC1: IC56.14(A)
ALU_CF_IN_SRC2: IC56.2(B)
ALU_CF_OUT_INV: IC58.1(A:I0)
ALU_MODE: IC14.8(M) IC15.8(M)
ALU_OP0: IC14.6(S0) IC15.6(S0) IC64.4(A:I2) IC157.1(A:I)
ALU_OP1: IC14.5(S1) IC15.5(S1) IC131.4(A:I2) IC151.1(A:I)
ALU_OP2: IC14.4(S2) IC15.4(S2) IC131.2(A:I1) IC150.1(A:I)
ALU_OP3: IC14.3(S3) IC15.3(S3) IC64.5(A:I3) IC158.1(A:I)
AUX_FLAGS_OUT: IC8.19(B:G) IC129.19(B:G)
AUX_FLAGS_WRT: IC128.1(M) IC128.2(N) IC144.1(M) IC144.2(N)
BH_OUT: IC124.19(B:G) IC125.19(B:G)
BH_WRT: IC153.1(G)
BL_OUT: IC2.19(B:G) IC3.19(B:G)
BL_WRT: IC100.1(G)
BPH_OUT: IC115.19(B:G) IC116.19(B:G)
BPH_WRT: IC99.1(G)
BPL_OUT: IC113.19(B:G) IC114.19(B:G)
BPL_WRT: IC98.1(G)
CF: IC46.5(2Q) IC59.5(2A) IC167.2(1A) IC195.13(B:A2)
CF_FROM_ALU: IC126.4(2D)
CH_OUT: IC154.19(B:G) IC155.19(B:G)
CH_WRT: IC185.1(G)
CL_OUT: IC102.19(B:G) IC117.19(B:G)
CL_WRT: IC101.1(G)
CLK: IC7.11(CLK) IC57.4(B:O) IC60.11(CLK) IC61.11(CLK) IC62.11(CLK) IC75.11(CLK) IC76.11(CLK) IC77.11(CLK) IC78.11(CLK) IC79.11(CLK) IC128.7(CLK) IC134.11(CLK) IC135.11(CLK) IC136.11(CLK) IC137.11(CLK) IC139.14(D1) IC144.7(CLK) IC162.11(CLK) IC189.11(CLK) IC248.7(CLK) IC249.7(CLK)
COND_0: IC142.14(A)
COND_1: IC142.2(B)
COND_2: IC73.1(!A!/B)
COND_SRC: IC59.1(!A!/B)
CONDITION: IC73.4(1Y) IC74.5(B:I1)
CPU_MEM_IO: IC60.6(Q3)
CPU_RD: IC60.2(Q1) IC69.11(B:A1)
CPU_WR: IC60.5(Q2) IC69.13(B:A2)
DATA0: IC20.3(D1) IC179.18(A:Y1)
DATA1: IC20.4(D2) IC179.16(A:Y2)
DATA2: IC20.7(D3) IC179.14(A:Y3)
DATA3: IC20.8(D4) IC179.12(A:Y4)
DATA4: IC20.13(D5) IC178.18(A:Y1)
DATA5: IC20.14(D6) IC178.16(A:Y2)
DATA6: IC20.17(D7) IC178.14(A:Y3)
DATA7: IC20.18(D8) IC178.12(A:Y4)
DH_OUT: IC145.19(B:G) IC146.19(B:G)
DH_WRT: IC184.1(G)
DL_OUT: IC186.19(B:G) IC215.19(B:G)
DMA_ACK: IC8.11(B:A1) IC144.3(Q1)
DMA_REQ: IC66.4(B:I0) IC162.4(D2) IC169.1(!A!/B) IC171.1(!A!/B) IC172.1(!A!/B) IC173.1(!A!/B)
DMA_TRISTATE: IC8.13(B:A2) IC28.19(B:G) IC29.19(B:G) IC69.19(B:G) IC70.19(B:G) IC71.19(B:G) IC144.4(Q2) IC250.4(B:I0) IC250.6(B:O)
FINAL_CONDITION: IC74.6(B:O) IC83.3(B:I)
FLAGS_REG_IN_SRC: IC47.1(!A!/B) IC210.1(!A!/B)
FLAGS_REG_OUT: IC195.19(B:G) IC196.19(B:G)
GND: IC22.15(G) IC23.15(G) IC34.4(1C2) IC34.12(2C2) IC40.4(1C2) IC40.12(2C2) IC41.4(1C2) IC41.12(2C2) IC47.15(G) IC49.5(2A) IC49.11(3A) IC49.14(4A) IC49.15(G) IC50.7(C0) IC53.11(B4) IC53.12(A4) IC53.14(A3) IC53.15(B3) IC55.2(1A) IC55.5(2A) IC55.11(3A) IC55.14(4A) IC55.15(G) IC56.1(1G) IC56.6(1C0) IC56.15(2G) IC59.15(G) IC63.2(1A) IC63.5(2A) IC63.11(3A) IC63.14(4A) IC63.15(G) IC68.2(1A) IC68.5(2A) IC68.10(3B) IC68.11(3A) IC68.13(4B) IC68.14(4A) IC68.15(G) IC69.17(B:A4) IC94.15(G) IC95.13(4B) IC95.15(G) IC96.15(G) IC97.15(G) IC118.8(A7) IC118.9(A8) IC119.15(G) IC121.15(G) IC128.9(G1) IC128.10(G2) IC139.9(G1) IC139.10(G2) IC144.9(G1) IC144.10(G2) IC160.17(B:A4) IC161.11(B:A1) IC161.13(B:A2) IC161.15(B:A3) IC161.17(B:A4) IC167.15(G) IC172.10(3B) IC172.11(3A) IC172.13(4B) IC172.14(4A) IC199.13(A:I4) IC210.5(2A) IC210.6(2B) IC210.10(3B) IC210.11(3A) IC210.13(4B) IC210.14(4A) IC210.15(G) IC217.2(A:A1) IC217.4(A:A2) IC217.6(A:A3) IC217.8(A:A4) IC217.11(B:A1) IC217.13(B:A2) IC217.15(B:A3) IC217.17(B:A4) IC226.5(EI) IC245.1(A:G) IC246.1(A:G) IC248.9(G1) IC248.10(G2) IC249.9(G1) IC249.10(G2) R4.1 R4.2 R4.3 R4.4 R4.5 R4.6 R4.7 R4.8 R5.1 R5.2 R5.3 R5.4 R5.5 R5.6 R5.7 R5.8 R6.9 R6.10 R6.11 R6.12 R6.13 R6.14 R6.15 R6.16 R7.1 R7.2 R7.3 R7.4 R7.5 R7.6 R7.7 R7.8 R8.1 R8.2 R8.3 R8.4 R8.5 R8.6 R8.7 R8.8 S1.2(P) S2.3(S) S4.3(S) U$1.1(A14) U$1.14(GND) U$1.20(/CE) U$1.22(/OE) U$1.27(/WE) U$2.1(A14) U$2.14(GND) U$2.20(/CE) U$2.22(/OE) U$2.27(/WE) U$3.1(A14) U$3.14(GND) U$3.20(/CE) U$3.22(/OE) U$3.27(/WE) U$4.1(A14) U$4.14(GND) U$4.20(/CE) U$4.22(/OE) U$4.27(/WE) U$5.1(A14) U$5.14(GND) U$5.20(/CE) U$5.22(/OE) U$5.27(/WE) U$6.1(A14) U$6.14(GND) U$6.20(/CE) U$6.22(/OE) U$6.27(/WE) U$7.1(A14) U$7.14(GND) U$7.20(/CE) U$7.22(/OE) U$7.27(/WE) U$8.1(A14) U$8.14(GND) U$8.20(/CE) U$8.22(/OE) U$8.27(/WE) U$9.1(A14) U$9.14(GND) U$9.20(/CE) U$9.22(/OE) U$9.27(/WE)
HALT: IC128.3(Q1) IC129.11(B:A1) IC147.5(B:I1)
IMM_X_OUT: IC217.1(A:G) IC217.19(B:G)
IMMY_OUT: IC19.1(A:G) IC19.19(B:G)
INT_ACK: IC222.4(G2A) IC222.5(G2B)
INT_ENABLE: IC8.15(B:A3) IC144.5(Q3) IC204.13(A:I2)
INT_PENDING: IC204.12(A:O)
INT_REQ: IC66.5(B:I1)
INT_REQ_0: IC163.3(A:CLK)
INT_REQ_1: IC164.3(A:CLK)
INT_REQ_2: IC168.3(A:CLK)
INT_REQ_3: IC174.3(A:CLK)
INT_REQ_4: IC188.3(A:CLK)
INT_REQ_5: IC221.3(A:CLK)
INT_STATUS_ENCODED_OUT: IC160.19(B:G) IC161.19(B:G)
INTERRUPT_STATUS_OUT: IC156.19(B:G) IC159.19(B:G)
IR_0: IC20.2(Q1) IC35.4(1C2)
IR_1: IC35.12(2C2)
IR_2: IC36.4(1C2)
IR_3: IC36.12(2C2)
IR_4: IC37.4(1C2)
IR_5: IC37.12(2C2)
IR_6: IC38.4(1C2)
IR_7: IC20.19(Q8) IC38.12(2C2)
MARH_WRT: IC7.1(G)
MARH_X_OUT: IC24.19(B:G) IC25.19(B:G)
MARL_0: IC27.11(B:A1) IC28.11(B:A1) IC189.2(1Q)
MARL_1: IC27.13(B:A2) IC28.13(B:A2) IC189.5(2Q)
MARL_WRT: IC189.1(G)
MARL_X_OUT: IC26.19(B:G) IC27.19(B:G)
MASK_0: IC201.9(C:I0) IC244.11(B:A1) IC248.3(Q1)
MASK_1: IC203.9(C:I0) IC244.13(B:A2) IC248.4(Q2)
MASK_2: IC206.9(C:I0) IC244.15(B:A3) IC248.5(Q3)
MASK_3: IC228.9(C:I0) IC244.17(B:A4) IC248.6(Q4)
MASK_4: IC190.9(C:I0) IC247.11(B:A1) IC249.3(Q1)
MASK_5: IC242.9(C:I0) IC247.13(B:A2) IC249.4(Q2)
MASK_ENABLE: IC8.17(B:A4) IC144.6(Q4) IC190.10(C:I1) IC201.10(C:I1) IC203.10(C:I1) IC206.10(C:I1) IC228.10(C:I1) IC242.10(C:I1)
MASK_FLAGS_OUT: IC244.19(B:G) IC247.19(B:G)
MASK_FLAGS_WRT: IC248.1(M) IC248.2(N) IC249.1(M) IC249.2(N)
MDR_IN_BUS0: IC21.3(1D) IC180.3(1D)
MDR_IN_BUS1: IC21.4(2D) IC180.4(2D)
MDR_IN_BUS2: IC21.7(3D) IC180.7(3D)
MDR_IN_BUS3: IC21.8(4D) IC180.8(4D)
MDR_IN_BUS4: IC21.13(5D) IC180.13(5D)
MDR_IN_BUS5: IC21.14(6D) IC180.14(6D)
MDR_IN_BUS6: IC21.17(7D) IC180.17(7D)
MDR_IN_BUS7: IC21.18(8D) IC180.18(8D)
MDR_IN_SRC: IC22.1(!A!/B) IC23.1(!A!/B)
MDRH_DATA_OUT: IC178.1(A:G) IC179.1(A:G)
MDRH_WRT: IC180.1(G)
MDRH_X_OUT: IC176.1(A:G) IC181.1(A:G)
MDRH_Y_OUT: IC182.1(A:G) IC183.1(A:G)
MDRL_DATA_OUT: IC30.1(A:G) IC31.1(A:G)
MDRL_WRT: IC21.1(G)
MDRL_X_OUT: IC12.1(A:G) IC13.1(A:G)
MDRL_Y_OUT: IC10.1(A:G) IC11.1(A:G)
MEM_IO: IC69.5(B:Y3) R10.6
N$1: IC1.2(1Q) IC9.2(A:A1)
N$2: IC1.5(2Q) IC9.4(A:A2)
N$3: IC1.6(3Q) IC9.6(A:A3)
N$4: IC1.9(4Q) IC9.8(A:A4)
N$5: IC1.12(5Q) IC9.11(B:A1)
N$6: IC1.15(6Q) IC9.13(B:A2)
N$7: IC1.16(7Q) IC9.15(B:A3)
N$8: IC1.19(8Q) IC9.17(B:A4)
N$9: IC139.1(M) IC139.2(N) IC147.6(B:O)
N$10: IC80.6(B:O) IC133.2(A:I1)
N$11: IC82.19(8Q) IC95.10(3B) IC104.9(A8)
N$12: IC49.4(1Y) IC50.6(B1)
N$13: IC2.11(B:A1) IC100.2(1Q)
N$14: IC49.7(2Y) IC50.2(B2)
N$15: IC2.13(B:A2) IC100.5(2Q)
N$16: IC2.15(B:A3) IC100.6(3Q)
N$17: IC2.17(B:A4) IC100.9(4Q)
N$18: IC3.11(B:A1) IC100.12(5Q)
N$19: IC3.13(B:A2) IC100.15(6Q)
N$20: IC3.15(B:A3) IC100.16(7Q)
N$21: IC3.17(B:A4) IC100.19(8Q)
N$22: IC56.3(1C3) IC57.2(A:O)
N$23: IC65.2(A:O) IC138.2(A:I1)
N$24: IC143.3(A:O) IC170.5(B:I1)
N$25: IC101.2(1Q) IC102.11(B:A1)
N$26: IC101.5(2Q) IC102.13(B:A2)
N$27: IC101.6(3Q) IC102.15(B:A3)
N$28: IC101.9(4Q) IC102.17(B:A4)
N$29: IC101.12(5Q) IC117.11(B:A1)
N$30: IC101.15(6Q) IC117.13(B:A2)
N$31: IC101.16(7Q) IC117.15(B:A3)
N$32: IC101.19(8Q) IC117.17(B:A4)
N$33: IC56.4(1C2) IC57.1(A:I) IC167.4(1Y)
N$34: IC160.15(B:A3)
N$35: IC49.9(3Y) IC50.15(B3)
N$36: IC49.12(4Y) IC50.11(B4)
N$37: IC51.6(B1) IC55.4(1Y)
N$38: IC51.2(B2) IC55.7(2Y)
N$39: IC51.15(B3) IC55.9(3Y)
N$40: IC51.11(B4) IC55.12(4Y)
N$41: IC160.13(B:A2)
N$42: IC179.2(A:A1) IC180.2(1Q) IC181.2(A:A1) IC182.2(A:A1)
N$43: IC179.4(A:A2) IC180.5(2Q) IC181.4(A:A2) IC182.4(A:A2)
N$44: IC179.6(A:A3) IC180.6(3Q) IC181.6(A:A3) IC182.6(A:A3)
N$45: IC179.8(A:A4) IC180.9(4Q) IC181.8(A:A4) IC182.8(A:A4)
N$46: IC176.2(A:A1) IC178.2(A:A1) IC180.12(5Q) IC183.2(A:A1)
N$47: IC176.4(A:A2) IC178.4(A:A2) IC180.15(6Q) IC183.4(A:A2)
N$48: IC176.6(A:A3) IC178.6(A:A3) IC180.16(7Q) IC183.6(A:A3)
N$49: IC128.4(Q2) IC129.13(B:A2)
N$50: IC130.6(B:O) IC141.1(A:I) IC143.2(A:I1)
N$51: IC176.8(A:A4) IC178.8(A:A4) IC180.19(8Q) IC183.8(A:A4)
N$52: IC27.15(B:A3) IC28.15(B:A3) IC189.6(3Q)
N$53: IC27.17(B:A4) IC28.17(B:A4) IC189.9(4Q)
N$54: IC26.11(B:A1) IC29.11(B:A1) IC189.12(5Q)
N$55: IC26.13(B:A2) IC29.13(B:A2) IC189.15(6Q)
N$56: IC26.15(B:A3) IC29.15(B:A3) IC189.16(7Q)
N$57: IC26.17(B:A4) IC29.17(B:A4) IC189.19(8Q)
N$58: IC7.2(1Q) IC25.11(B:A1) IC70.11(B:A1)
N$59: IC7.5(2Q) IC25.13(B:A2) IC70.13(B:A2)
N$60: IC7.6(3Q) IC25.15(B:A3) IC70.15(B:A3)
N$61: IC7.9(4Q) IC25.17(B:A4) IC70.17(B:A4)
N$62: IC7.12(5Q) IC24.11(B:A1) IC71.11(B:A1)
N$63: IC7.15(6Q) IC24.13(B:A2) IC71.13(B:A2)
N$64: IC7.16(7Q) IC24.15(B:A3) IC71.15(B:A3)
N$65: IC52.6(B1) IC63.4(1Y)
N$66: IC46.19(8Q) IC196.17(B:A4)
N$67: IC5.2(1Q) IC109.11(B:A1)
N$68: IC5.5(2Q) IC109.13(B:A2)
N$69: IC5.6(3Q) IC109.15(B:A3)
N$70: IC5.9(4Q) IC109.17(B:A4)
N$71: IC5.12(5Q) IC110.11(B:A1)
N$72: IC5.15(6Q) IC110.13(B:A2)
N$73: IC7.19(8Q) IC24.17(B:A4) IC71.17(B:A4)
N$74: IC52.2(B2) IC63.7(2Y)
N$75: IC52.15(B3) IC63.9(3Y)
N$76: IC44.3(A:CLK) IC139.7(CLK) SW3.C
N$77: IC75.3(D1) U$1.11(I/O0)
N$78: IC39.1(A:I0) IC43.4(B:O) IC45.1(A:I0)
N$79: IC73.3(1B) IC142.9(2Y)
N$80: IC83.4(B:O)
N$81: IC138.1(A:I0) IC141.2(A:O)
N$82: IC138.3(A:O) IC170.4(B:I0)
N$83: IC10.2(A:A1) IC13.2(A:A1) IC21.2(1Q) IC30.2(A:A1)
N$84: IC133.1(A:I0) IC170.6(B:O)
N$85: IC64.6(A:O) IC65.1(A:I)
N$86: IC64.2(A:I1) IC150.2(A:O)
N$87: IC145.11(B:A1) IC184.2(1Q)
N$88: IC64.1(A:I0) IC151.2(A:O)
N$89: IC131.6(A:O) IC132.1(A:I)
N$90: IC132.2(A:O) IC143.1(A:I0)
N$91: IC14.2(A0) R5.16
N$92: IC14.23(A1) R5.15
N$93: IC14.21(A2) R5.14
N$94: IC14.19(A3) R5.13
N$95: IC15.2(A0) R5.12
N$96: IC15.23(A1) R5.11
N$97: IC15.21(A2) R5.10
N$98: IC15.19(A3) R5.9
N$99: IC14.1(B0) R4.9
N$100: IC14.22(B1) R4.10
N$101: IC14.20(B2) R4.11
N$102: IC14.18(B3) R4.12
N$103: IC11.12(A:Y4) IC15.1(B0) R4.13
N$104: IC11.14(A:Y3) IC15.22(B1) R4.14
N$105: IC11.16(A:Y2) IC15.20(B2) R4.15
N$106: IC11.18(A:Y1) IC15.18(B3) R4.16
N$107: IC14.16(CN+4) IC15.7(CN)
N$108: IC46.4(2D) IC47.7(2Y)
N$109: IC145.13(B:A2) IC184.5(2Q)
N$110: IC131.5(A:I3) IC157.2(A:O)
N$111: IC145.15(B:A3) IC184.6(3Q)
N$112: IC145.17(B:A4) IC184.9(4Q)
N$113: IC131.1(A:I0) IC158.2(A:O)
N$114: IC86.2(1Q) IC89.2(A:A1)
N$115: IC86.5(2Q) IC89.4(A:A2)
N$116: IC86.6(3Q) IC89.6(A:A3)
N$117: IC86.9(4Q) IC89.8(A:A4)
N$118: IC86.12(5Q) IC90.2(A:A1)
N$119: IC86.15(6Q) IC90.4(A:A2)
N$120: IC86.16(7Q) IC90.6(A:A3)
N$121: IC86.19(8Q) IC90.8(A:A4)
N$122: IC88.2(1Q) IC91.2(A:A1)
N$123: IC88.5(2Q) IC91.4(A:A2)
N$124: IC88.6(3Q) IC91.6(A:A3)
N$125: IC88.9(4Q) IC91.8(A:A4)
N$126: IC88.12(5Q) IC92.2(A:A1)
N$127: IC88.15(6Q) IC92.4(A:A2)
N$128: IC88.16(7Q) IC92.6(A:A3)
N$129: IC88.19(8Q) IC92.8(A:A4)
N$130: IC42.2(A:I1) IC67.6(B:O)
N$131: IC93.3(1D) IC96.4(1Y)
N$132: IC10.4(A:A2) IC13.4(A:A2) IC21.5(2Q) IC30.4(A:A2)
N$133: IC45.3(A:O) IC67.5(B:I1)
N$134: IC10.6(A:A3) IC13.6(A:A3) IC21.6(3Q) IC30.6(A:A3)
N$135: IC146.11(B:A1) IC184.12(5Q)
N$136: IC146.13(B:A2) IC184.15(6Q)
N$137: IC10.8(A:A4) IC13.8(A:A4) IC21.9(4Q) IC30.8(A:A4)
N$138: IC11.2(A:A1) IC12.2(A:A1) IC21.12(5Q) IC31.2(A:A1)
N$139: IC146.15(B:A3) IC184.16(7Q)
N$140: IC11.4(A:A2) IC12.4(A:A2) IC21.15(6Q) IC31.4(A:A2)
N$141: IC11.6(A:A3) IC12.6(A:A3) IC21.16(7Q) IC31.6(A:A3)
N$142: IC146.17(B:A4) IC184.19(8Q)
N$143: IC5.16(7Q) IC110.15(B:A3)
N$144: IC52.11(B4) IC63.12(4Y)
N$145: IC53.6(B1) IC68.4(1Y)
N$146: IC5.19(8Q) IC110.17(B:A4)
N$147: IC53.2(B2) IC68.7(2Y)
N$148: IC93.4(2D) IC96.7(2Y)
N$149: IC93.7(3D) IC96.9(3Y)
N$150: IC55.13(4B) IC63.3(1B) IC63.6(2B) IC63.10(3B) IC63.13(4B) IC68.3(1B) IC68.6(2B)
N$151: IC4.2(1Q) IC111.11(B:A1)
N$152: IC49.1(!A!/B) IC55.1(!A!/B) IC63.1(!A!/B) IC68.1(!A!/B) IC85.12(A:O)
N$153: IC45.2(A:I1) IC66.6(B:O)
N$154: IC84.4(B:O)
N$155: IC128.5(Q3) IC129.15(B:A3)
N$156: IC93.8(4D) IC96.12(4Y)
N$157: IC93.13(5D) IC94.4(1Y)
N$158: IC93.14(6D) IC94.7(2Y)
N$159: IC93.17(7D) IC94.9(3Y)
N$160: IC93.18(8D) IC94.12(4Y)
N$161: IC82.3(1D) IC97.4(1Y)
N$162: IC82.4(2D) IC97.7(2Y)
N$163: IC82.7(3D) IC97.9(3Y)
N$164: IC11.8(A:A4) IC12.8(A:A4) IC21.19(8Q) IC31.8(A:A4)
N$165: IC82.8(4D) IC97.12(4Y)
N$166: IC82.13(5D) IC95.4(1Y)
N$167: SW3.2
N$168: IC82.14(6D) IC95.7(2Y)
N$169: IC10.18(A:Y1)
N$170: IC10.16(A:Y2)
N$171: IC10.14(A:Y3)
N$172: IC10.12(A:Y4)
N$173: IC82.17(7D) IC95.9(3Y)
N$174: R7.9 SW1.8
N$175: IC47.5(2A) IC58.3(A:O)
N$176: IC14.7(CN) IC56.7(1Y)
N$177: IC13.18(A:Y1)
N$178: IC13.16(A:Y2)
N$179: IC13.14(A:Y3)
N$180: IC13.12(A:Y4)
N$181: IC12.18(A:Y1)
N$182: IC12.16(A:Y2)
N$183: IC12.14(A:Y3)
N$184: IC12.12(A:Y4)
N$185: IC47.2(1A) IC119.4(1Y)
N$186: R7.10 SW1.7
N$187: R7.11 SW1.6
N$188: R7.12 SW1.5
N$189: R7.13 SW1.4
N$190: R7.14 SW1.3
N$191: IC22.7(2Y)
N$192: IC22.9(3Y)
N$193: IC22.12(4Y)
N$194: IC23.4(1Y)
N$195: IC23.7(2Y)
N$196: IC23.9(3Y)
N$197: IC23.12(4Y)
N$198: IC22.3(1B)
N$199: IC22.6(2B)
N$200: IC30.18(A:Y1)
N$201: IC30.16(A:Y2)
N$202: IC82.18(8D) IC95.12(4Y)
N$203: IC30.14(A:Y3)
N$204: IC30.12(A:Y4)
N$205: IC82.16(7Q) IC95.6(2B) IC104.8(A7)
N$206: IC31.18(A:Y1)
N$207: IC31.16(A:Y2)
N$208: IC31.14(A:Y3)
N$209: IC31.12(A:Y4)
N$210: IC22.4(1Y)
N$211: IC22.10(3B)
N$212: IC22.13(4B)
N$213: IC23.3(1B)
N$214: IC23.6(2B)
N$215: IC23.10(3B)
N$216: IC23.13(4B)
N$217: IC128.6(Q4) IC129.17(B:A4)
N$218: IC46.7(3D) IC47.9(3Y)
N$219: IC46.8(4D) IC47.12(4Y)
N$220: R7.15 SW1.2
N$221: IC122.11(B:A1) IC123.12(5Q)
N$222: R6.8 SW2.1
N$223: R6.7 SW2.2
N$224: R6.6 SW2.3
N$225: R6.5 SW2.4
N$226: R6.4 SW2.5
N$227: R6.3 SW2.6
N$228: R6.2 SW2.7
N$229: IC122.13(B:A2) IC123.15(6Q)
N$230: IC122.15(B:A3) IC123.16(7Q)
N$231: IC119.3(1B) IC120.3(A:O)
N$232: IC82.15(6Q) IC95.3(1B) IC104.7(A6)
N$233: IC82.12(5Q) IC97.13(4B) IC104.6(A5)
N$235: IC122.17(B:A4) IC123.19(8Q)
N$236: IC122.2(A:A1) IC123.2(1Q)
N$237: IC122.4(A:A2) IC123.5(2Q)
N$238: IC122.6(A:A3) IC123.6(3Q)
N$239: IC32.3(D1) IC41.7(1Y)
N$240: IC32.11(CLK) IC33.11(CLK)
N$241: IC32.1(CLR) IC33.1(CLR)
N$242: IC32.4(D2) IC41.9(2Y)
N$243: IC32.7(D3) IC40.7(1Y)
N$244: IC32.8(D4) IC40.9(2Y)
N$245: IC32.13(D5) IC34.7(1Y)
N$246: IC32.14(D6) IC34.9(2Y)
N$247: IC33.3(D1) IC35.7(1Y)
N$248: IC33.4(D2) IC35.9(2Y)
N$249: IC122.8(A:A4) IC123.9(4Q)
N$250: IC33.7(D3) IC36.7(1Y)
N$251: U$2.10(A0)
N$252: U$2.9(A1)
N$253: U$2.8(A2)
N$254: U$2.7(A3)
N$255: U$2.6(A4)
N$256: U$2.5(A5)
N$257: U$2.4(A6)
N$258: U$2.3(A7)
N$259: U$2.25(A8)
N$260: U$2.24(A9)
N$261: U$2.21(A10)
N$262: U$2.23(A11)
N$263: U$2.2(A12)
N$264: U$2.26(A13)
N$265: U$3.10(A0)
N$266: U$3.9(A1)
N$267: U$3.8(A2)
N$268: U$3.7(A3)
N$269: U$3.6(A4)
N$270: U$3.5(A5)
N$271: U$3.4(A6)
N$272: U$3.3(A7)
N$273: U$3.25(A8)
N$274: U$3.24(A9)
N$275: U$3.21(A10)
N$276: U$3.23(A11)
N$277: U$3.2(A12)
N$278: U$3.26(A13)
N$279: U$4.10(A0)
N$280: U$4.9(A1)
N$281: U$4.8(A2)
N$282: U$4.7(A3)
N$283: U$4.6(A4)
N$284: U$4.5(A5)
N$285: U$4.4(A6)
N$286: U$4.3(A7)
N$287: U$4.25(A8)
N$288: U$4.24(A9)
N$289: U$4.21(A10)
N$290: U$4.23(A11)
N$291: U$4.2(A12)
N$292: U$4.26(A13)
N$293: U$5.10(A0)
N$294: U$5.9(A1)
N$295: U$5.8(A2)
N$296: U$5.7(A3)
N$297: U$5.6(A4)
N$298: U$5.5(A5)
N$299: U$5.4(A6)
N$300: U$5.3(A7)
N$301: U$5.25(A8)
N$302: U$5.24(A9)
N$303: U$5.21(A10)
N$304: U$5.23(A11)
N$305: U$5.2(A12)
N$306: U$5.26(A13)
N$307: IC33.8(D4) IC36.9(2Y)
N$308: IC33.13(D5) IC37.7(1Y)
N$309: IC33.14(D6) IC37.9(2Y)
N$310: IC33.17(D7) IC38.7(1Y)
N$311: IC33.18(D8) IC38.9(2Y)
N$312: IC82.9(4Q) IC97.10(3B) IC104.5(A4)
N$313: IC82.6(3Q) IC97.6(2B) IC104.4(A3)
N$314: IC82.5(2Q) IC97.3(1B) IC104.3(A2)
N$315: IC82.2(1Q) IC94.13(4B) IC104.2(A1)
N$316: IC93.19(8Q) IC94.10(3B) IC103.9(A8)
N$317: IC93.16(7Q) IC94.6(2B) IC103.8(A7)
N$318: IC93.15(6Q) IC94.3(1B) IC103.7(A6)
N$319: IC93.12(5Q) IC96.13(4B) IC103.6(A5)
N$320: IC226.9(A0)
N$321: IC93.9(4Q) IC96.10(3B) IC103.5(A4)
N$322: IC175.6(B:O) IC177.4(B:I0)
N$323: IC93.6(3Q) IC96.6(2B) IC103.4(A3)
N$324: IC177.6(B:O) IC192.4(B:I0)
N$325: IC124.11(B:A1) IC153.2(1Q)
N$326: IC124.13(B:A2) IC153.5(2Q)
N$327: IC124.15(B:A3) IC153.6(3Q)
N$328: IC124.17(B:A4) IC153.9(4Q)
N$329: IC125.11(B:A1) IC153.12(5Q)
N$330: IC125.13(B:A2) IC153.15(6Q)
N$331: IC125.15(B:A3) IC153.16(7Q)
N$332: IC125.17(B:A4) IC153.19(8Q)
N$333: IC50.5(A1)
N$334: IC50.3(A2)
N$335: IC50.14(A3)
N$336: IC50.12(A4)
N$337: IC52.5(A1)
N$338: IC51.5(A1)
N$339: IC51.3(A2)
N$340: IC51.14(A3)
N$341: IC51.12(A4)
N$342: IC154.11(B:A1) IC185.2(1Q)
N$343: IC93.5(2Q) IC96.3(1B) IC103.3(A2)
N$344: IC93.2(1Q) IC103.2(A1)
N$345: IC121.4(1Y) IC126.3(1D)
N$346: IC190.8(C:O) IC191.1(A:I0)
N$347: IC121.3(1B) IC127.3(A:O)
N$348: IC148.3(B:I) IC156.11(B:A1) IC162.2(Q1)
N$349: IC149.3(B:I) IC226.14(GS)
N$350: IC52.3(A2)
N$351: IC52.14(A3)
N$352: IC52.12(A4)
N$353: IC53.5(A1)
N$354: IC53.3(A2)
N$355: IC191.3(A:O) IC226.11
N$356: IC149.4(B:O) IC204.2(A:I1)
N$357: IC50.9(C4) IC51.7(C0)
N$358: IC51.9(C4) IC52.7(C0)
N$359: IC52.9(C4) IC53.7(C0)
N$360: IC76.5(Q2)
N$361: IC204.1(A:I0) IC226.15(EO)
N$362: IC192.6(B:O) IC193.4(B:I0)
N$363: IC148.4(B:O) IC226.4
N$364: IC76.6(Q3)
N$365: IC152.4(B:O) IC226.3
N$366: IC152.3(B:I) IC156.13(B:A2) IC162.5(Q2)
N$367: IC75.4(D2) U$1.12(I/O1)
N$368: IC201.8(C:O) IC202.1(A:I0)
N$369: IC75.7(D3) U$1.13(I/O2)
N$370: IC46.3(1D) IC47.4(1Y)
N$371: IC15.16(CN+4) IC58.2(A:I1)
N$372: IC168.1(A:CLR) IC220.3(A:O)
N$373: IC154.13(B:A2) IC185.5(2Q)
N$374: IC174.1(A:CLR) IC223.3(A:O)
N$375: IC75.8(D4) U$1.15(I/O3)
N$376: IC75.13(D5) U$1.16(I/O4)
N$377: IC75.14(D6) U$1.17(I/O5)
N$378: IC60.3(D1) U$10.11(I/O0)
N$379: IC60.4(D2) U$10.12(I/O1)
N$380: IC60.7(D3) U$10.13(I/O2)
N$381: IC60.8(D4) U$10.15(I/O3)
N$382: IC60.13(D5) U$10.16(I/O4)
N$383: IC60.14(D6) U$10.17(I/O5)
N$384: IC60.17(D7) U$10.18(I/O6)
N$385: IC60.18(D8) U$10.19(I/O7)
N$386: IC61.3(D1) U$11.11(I/O0)
N$387: IC61.4(D2) U$11.12(I/O1)
N$388: IC188.1(A:CLR) IC224.3(A:O)
N$389: IC162.3(D1) IC207.3(A:O)
N$390: IC162.7(D3) IC163.5(A:Q)
N$391: IC76.9(Q4)
N$392: IC162.8(D4) IC164.5(A:Q)
N$393: IC162.13(D5) IC168.5(A:Q)
N$394: IC162.14(D6) IC174.5(A:Q)
N$395: IC162.17(D7) IC188.5(A:Q)
N$396: IC162.18(D8) IC221.5(A:Q)
N$397: IC208.2(A:I1) IC222.15(Y0)
N$398: IC218.2(A:I1) IC222.13(Y2)
N$399: IC219.2(A:I1) IC222.12(Y3)
N$400: IC76.12(Q5)
N$401: IC76.15(Q6)
N$402: IC76.16(Q7)
N$403: IC222.10(Y5) IC223.1(A:I0)
N$404: IC4.5(2Q) IC111.13(B:A2)
N$405: IC222.7(Y7) IC225.1(A:I0)
N$406: IC187.5(A:Q) IC207.2(A:I1)
N$407: IC187.1(A:CLR) IC208.3(A:O)
N$408: IC163.1(A:CLR) IC218.3(A:O)
N$409: IC164.1(A:CLR) IC219.3(A:O)
N$410: IC221.1(A:CLR) IC225.3(A:O)
N$411: IC156.15(B:A3) IC162.6(Q3) IC202.2(A:I1)
N$412: IC156.17(B:A4) IC162.9(Q4) IC205.2(A:I1)
N$413: IC202.3(A:O) IC226.2
N$414: IC159.11(B:A1) IC162.12(Q5) IC227.2(A:I1)
N$415: IC203.8(C:O) IC205.1(A:I0)
N$416: IC205.3(A:O) IC226.1
N$417: IC206.8(C:O) IC227.1(A:I0)
N$418: IC226.13 IC227.3(A:O)
N$419: IC228.8(C:O) IC241.1(A:I0)
N$420: IC226.12 IC241.3(A:O)
N$421: IC242.8(C:O) IC243.1(A:I0)
N$422: IC154.15(B:A3) IC185.6(3Q)
N$423: IC154.17(B:A4) IC185.9(4Q)
N$424: IC155.11(B:A1) IC185.12(5Q)
N$425: IC155.13(B:A2) IC185.15(6Q)
N$426: IC155.15(B:A3) IC185.16(7Q)
N$427: IC155.17(B:A4) IC185.19(8Q)
N$428: IC186.11(B:A1) IC216.2(1Q)
N$429: IC186.13(B:A2) IC216.5(2Q)
N$430: IC186.15(B:A3) IC216.6(3Q)
N$431: IC186.17(B:A4) IC216.9(4Q)
N$432: IC215.11(B:A1) IC216.12(5Q)
N$433: IC215.13(B:A2) IC216.15(6Q)
N$434: IC215.15(B:A3) IC216.16(7Q)
N$435: IC215.17(B:A4) IC216.19(8Q)
N$436: IC226.10 IC243.3(A:O)
N$437: IC159.13(B:A2) IC162.15(Q6) IC241.2(A:I1)
N$438: IC159.15(B:A3) IC162.16(Q7) IC191.2(A:I1)
N$439: IC159.17(B:A4) IC162.19(Q8) IC243.2(A:I1)
N$440: IC76.19(Q8)
N$441: IC247.15(B:A3) IC249.5(Q3)
N$442: IC76.3(D1) U$2.11(I/O0)
N$443: IC76.4(D2) U$2.12(I/O1)
N$444: IC247.17(B:A4) IC249.6(Q4)
N$445: IC193.6(B:O) IC194.4(B:I0)
N$446: IC197.5(A:O) IC198.1(A:I)
N$447: IC77.5(Q2)
N$448: IC61.7(D3) U$11.13(I/O2)
N$449: IC75.17(D7) U$1.18(I/O6)
N$450: IC75.18(D8) U$1.19(I/O7)
N$451: IC76.7(D3) U$2.13(I/O2)
N$452: IC76.8(D4) U$2.15(I/O3)
N$453: IC76.13(D5) U$2.16(I/O4)
N$454: IC76.14(D6) U$2.17(I/O5)
N$455: IC76.17(D7) U$2.18(I/O6)
N$456: IC76.18(D8) U$2.19(I/O7)
N$457: IC77.3(D1) U$3.11(I/O0)
N$458: IC77.4(D2) U$3.12(I/O1)
N$459: IC77.7(D3) U$3.13(I/O2)
N$460: IC77.8(D4) U$3.15(I/O3)
N$461: IC77.13(D5) U$3.16(I/O4)
N$462: IC77.14(D6) U$3.17(I/O5)
N$463: IC77.17(D7) U$3.18(I/O6)
N$464: IC77.18(D8) U$3.19(I/O7)
N$465: IC78.3(D1) U$4.11(I/O0)
N$466: IC78.4(D2) U$4.12(I/O1)
N$467: IC78.7(D3) U$4.13(I/O2)
N$468: IC78.8(D4) U$4.15(I/O3)
N$469: IC78.13(D5) U$4.16(I/O4)
N$470: IC78.14(D6) U$4.17(I/O5)
N$471: IC78.17(D7) U$4.18(I/O6)
N$472: IC78.18(D8) U$4.19(I/O7)
N$473: IC79.3(D1) U$5.11(I/O0)
N$474: IC79.4(D2) U$5.12(I/O1)
N$475: IC79.7(D3) U$5.13(I/O2)
N$476: IC79.8(D4) U$5.15(I/O3)
N$477: IC79.13(D5) U$5.16(I/O4)
N$478: IC79.14(D6) U$5.17(I/O5)
N$479: IC79.17(D7) U$5.18(I/O6)
N$480: IC79.18(D8) U$5.19(I/O7)
N$481: IC198.2(A:O) IC199.1(A:I0)
N$482: IC61.8(D4) U$11.15(I/O3)
N$483: IC61.13(D5) U$11.16(I/O4)
N$484: IC61.14(D6) U$11.17(I/O5)
N$485: IC61.17(D7) U$11.18(I/O6)
N$486: IC61.18(D8) U$11.19(I/O7)
N$487: IC62.3(D1) U$12.11(I/O0)
N$488: IC62.4(D2) U$12.12(I/O1)
N$489: IC62.7(D3) U$12.13(I/O2)
N$490: IC62.8(D4) U$12.15(I/O3)
N$491: IC62.13(D5) U$12.16(I/O4)
N$492: IC62.14(D6) U$12.17(I/O5)
N$493: IC62.17(D7) U$12.18(I/O6)
N$494: IC62.18(D8) U$12.19(I/O7)
N$495: IC194.6(B:O) IC200.4(B:I0)
N$496: IC200.6(B:O) IC209.4(B:I0)
N$497: IC46.13(5D) IC210.4(1Y)
N$498: IC46.14(6D) IC210.7(2Y)
N$499: IC46.17(7D) IC210.9(3Y)
N$500: IC46.18(8D) IC210.12(4Y)
N$503: IC134.18(D8) U$6.19(I/O7)
N$504: IC134.17(D7) U$6.18(I/O6)
N$505: IC134.14(D6) U$6.17(I/O5)
N$506: IC134.13(D5) U$6.16(I/O4)
N$507: IC134.8(D4) U$6.15(I/O3)
N$508: IC134.7(D3) U$6.13(I/O2)
N$509: IC134.4(D2) U$6.12(I/O1)
N$510: IC134.3(D1) U$6.11(I/O0)
N$511: IC135.3(D1) U$7.11(I/O0)
N$512: IC135.4(D2) U$7.12(I/O1)
N$513: IC135.7(D3) U$7.13(I/O2)
N$514: IC135.8(D4) U$7.15(I/O3)
N$515: IC135.13(D5) U$7.16(I/O4)
N$516: IC135.14(D6) U$7.17(I/O5)
N$517: IC135.17(D7) U$7.18(I/O6)
N$518: IC135.18(D8) U$7.19(I/O7)
N$519: IC136.3(D1) U$8.11(I/O0)
N$520: IC136.4(D2) U$8.12(I/O1)
N$521: IC136.7(D3) U$8.13(I/O2)
N$522: IC136.8(D4) U$8.15(I/O3)
N$523: IC136.13(D5) U$8.16(I/O4)
N$524: IC136.14(D6) U$8.17(I/O5)
N$525: IC136.17(D7) U$8.18(I/O6)
N$526: IC136.18(D8) U$8.19(I/O7)
N$527: IC137.3(D1) U$9.11(I/O0)
N$528: IC87.3(A:S2) R1.1 S1.1(O)
N$529: IC87.1(A:R) R2.1 S1.3(S)
N$531: IC87.4(A:Q) SW3.1
N$532: SW3.4
N$533: IC137.4(D2) U$9.12(I/O1)
N$534: IC137.7(D3) U$9.13(I/O2)
N$535: IC137.8(D4) U$9.15(I/O3)
N$536: IC137.13(D5) U$9.16(I/O4)
N$537: IC137.14(D6) U$9.17(I/O5)
N$538: IC137.17(D7) U$9.18(I/O6)
N$539: IC137.18(D8) U$9.19(I/O7)
N$548: IC57.3(B:I) IC139.3(Q1)
N$558: IC73.2(1A) IC142.7(1Y)
N$564: IC77.6(Q3)
N$567: IC81.6(B:O) IC142.12(2C2)
N$568: IC77.9(Q4)
N$569: IC18.6(B:O) IC142.13(2C3)
N$571: IC77.12(Q5)
N$574: IC16.2(1Q) IC211.2(A:A1)
N$575: IC16.5(2Q) IC211.4(A:A2)
N$576: IC16.6(3Q) IC211.6(A:A3)
N$577: IC4.6(3Q) IC111.15(B:A3)
N$578: IC4.9(4Q) IC111.17(B:A4)
N$579: IC4.12(5Q) IC112.11(B:A1)
N$580: IC4.15(6Q) IC112.13(B:A2)
N$581: IC4.16(7Q) IC112.15(B:A3)
N$582: IC4.19(8Q) IC112.17(B:A4)
N$583: IC98.2(1Q) IC113.11(B:A1)
N$584: IC98.5(2Q) IC113.13(B:A2)
N$585: IC98.6(3Q) IC113.15(B:A3)
N$586: IC98.9(4Q) IC113.17(B:A4)
N$587: IC98.12(5Q) IC114.11(B:A1)
N$588: IC98.15(6Q) IC114.13(B:A2)
N$589: IC98.16(7Q) IC114.15(B:A3)
N$590: IC98.19(8Q) IC114.17(B:A4)
N$591: IC99.2(1Q) IC115.11(B:A1)
N$592: IC99.5(2Q) IC115.13(B:A2)
N$593: IC99.6(3Q) IC115.15(B:A3)
N$594: IC99.9(4Q) IC115.17(B:A4)
N$595: IC99.12(5Q) IC116.11(B:A1)
N$596: IC99.15(6Q) IC116.13(B:A2)
N$597: IC99.16(7Q) IC116.15(B:A3)
N$598: IC99.19(8Q) IC116.17(B:A4)
N$601: IC16.9(4Q) IC211.8(A:A4)
N$602: IC77.15(Q6)
N$603: IC16.12(5Q) IC212.2(A:A1)
N$604: IC16.15(6Q) IC212.4(A:A2)
N$605: IC77.16(Q7)
N$606: IC77.19(Q8)
N$607: IC78.2(Q1)
N$608: IC78.5(Q2)
N$609: IC78.6(Q3)
N$610: IC78.9(Q4)
N$611: IC78.12(Q5)
N$612: IC78.15(Q6)
N$613: IC78.16(Q7)
N$614: IC78.19(Q8)
N$615: IC79.2(Q1)
N$616: IC79.5(Q2)
N$617: IC79.6(Q3)
N$618: IC79.9(Q4)
N$619: IC79.12(Q5)
N$620: IC79.15(Q6)
N$621: IC79.16(Q7)
N$622: IC79.19(Q8)
N$623: IC134.2(Q1)
N$624: IC134.5(Q2)
N$625: IC134.6(Q3)
N$626: IC134.9(Q4)
N$627: IC134.12(Q5)
N$628: IC134.15(Q6)
N$629: IC134.16(Q7)
N$630: IC134.19(Q8)
N$631: IC135.2(Q1)
N$632: IC135.5(Q2)
N$633: IC135.6(Q3)
N$634: IC135.9(Q4)
N$635: IC135.12(Q5)
N$636: IC135.15(Q6)
N$637: IC135.16(Q7)
N$638: IC135.19(Q8)
N$639: IC136.2(Q1)
N$640: IC136.5(Q2)
N$641: IC136.6(Q3)
N$642: IC136.9(Q4)
N$643: IC136.12(Q5)
N$644: IC136.15(Q6)
N$645: IC136.16(Q7)
N$646: IC136.19(Q8)
N$647: IC137.2(Q1)
N$648: IC137.5(Q2)
N$649: IC137.6(Q3)
N$650: IC137.9(Q4)
N$651: IC137.12(Q5)
N$652: IC137.15(Q6)
N$653: IC137.16(Q7)
N$654: IC137.19(Q8)
N$655: IC16.16(7Q) IC212.6(A:A3)
N$656: IC16.19(8Q) IC212.8(A:A4)
N$657: IC17.2(1Q) IC213.2(A:A1)
N$658: IC17.5(2Q) IC213.4(A:A2)
N$659: IC17.6(3Q) IC213.6(A:A3)
N$660: IC17.9(4Q) IC213.8(A:A4)
N$661: IC17.12(5Q) IC214.2(A:A1)
N$662: IC17.15(6Q) IC214.4(A:A2)
N$663: IC17.16(7Q) IC214.6(A:A3)
N$664: IC17.19(8Q) IC214.8(A:A4)
N$685: IC220.1(A:I0) IC222.11(Y4)
N$686: IC14.9(F0) IC245.2(A:A1)
N$687: IC222.9(Y6) IC224.1(A:I0)
N$688: IC229.2(A:A1) IC234.2(1Q)
N$689: IC229.4(A:A2) IC234.5(2Q)
N$690: IC229.6(A:A3) IC234.6(3Q)
N$691: IC230.2(A:A1) IC234.12(5Q)
N$692: IC230.4(A:A2) IC234.15(6Q)
N$693: IC230.6(A:A3) IC234.16(7Q)
N$694: IC230.8(A:A4) IC234.19(8Q)
N$695: IC231.2(A:A1) IC233.2(1Q)
N$696: IC231.4(A:A2) IC233.5(2Q)
N$697: IC231.6(A:A3) IC233.6(3Q)
N$698: IC231.8(A:A4) IC233.9(4Q)
N$699: IC232.2(A:A1) IC233.12(5Q)
N$700: IC232.4(A:A2) IC233.15(6Q)
N$701: IC232.6(A:A3) IC233.16(7Q)
N$702: IC232.8(A:A4) IC233.19(8Q)
N$703: IC230.1(A:G)
N$704: IC234.9(4Q)
N$705: IC235.2(A:A1) IC240.2(1Q)
N$706: IC235.4(A:A2) IC240.5(2Q)
N$707: IC235.6(A:A3) IC240.6(3Q)
N$708: IC236.2(A:A1) IC240.12(5Q)
N$709: IC236.4(A:A2) IC240.15(6Q)
N$710: IC236.6(A:A3) IC240.16(7Q)
N$711: IC236.8(A:A4) IC240.19(8Q)
N$712: IC237.2(A:A1) IC239.2(1Q)
N$713: IC237.4(A:A2) IC239.5(2Q)
N$714: IC237.6(A:A3) IC239.6(3Q)
N$715: IC237.8(A:A4) IC239.9(4Q)
N$716: IC238.2(A:A1) IC239.12(5Q)
N$717: IC238.4(A:A2) IC239.15(6Q)
N$718: IC238.6(A:A3) IC239.16(7Q)
N$719: IC238.8(A:A4) IC239.19(8Q)
N$720: IC236.1(A:G)
N$721: IC240.9(4Q)
NOT_CONDITION: IC74.4(B:I0)
NOT_RST: IC20.1(CLR) IC75.1(CLR) IC76.1(CLR) IC77.1(CLR) IC78.1(CLR) IC79.1(CLR) IC134.1(CLR) IC135.1(CLR) IC136.1(CLR) IC137.1(CLR)
OF: IC46.9(4Q) IC59.14(4A) IC195.17(B:A4)
OF_FROM_ALU: IC47.14(4A) IC126.8(4D)
PANEL_MEM_IO: R10.11
PANEL_RD: R10.9
PANEL_WR: R10.10
PCH_0: IC6.2(1Q) IC107.11(B:A1)
PCH_1: IC6.5(2Q) IC107.13(B:A2)
PCH_2: IC6.6(3Q) IC107.15(B:A3)
PCH_3: IC6.9(4Q) IC107.17(B:A4)
PCH_4: IC6.12(5Q) IC108.11(B:A1)
PCH_5: IC6.15(6Q) IC108.13(B:A2)
PCH_6: IC6.16(7Q) IC108.15(B:A3)
PCH_7: IC6.19(8Q) IC108.17(B:A4)
PCH_OUT: IC107.19(B:G) IC108.19(B:G)
PCH_WRT: IC6.1(G)
PCL_0: IC48.2(1Q) IC105.11(B:A1)
PCL_1: IC48.5(2Q) IC105.13(B:A2)
PCL_2: IC48.6(3Q) IC105.15(B:A3)
PCL_3: IC48.9(4Q) IC105.17(B:A4)
PCL_4: IC48.12(5Q) IC106.11(B:A1)
PCL_5: IC48.15(6Q) IC106.13(B:A2)
PCL_6: IC48.16(7Q) IC106.15(B:A3)
PCL_7: IC48.19(8Q) IC106.17(B:A4)
PCL_OUT: IC105.19(B:G) IC106.19(B:G)
PCL_WRT: IC48.1(G)
PF: IC46.12(5Q) IC142.10(2C0) IC196.11(B:A1)
PF_FROM_ALU: IC209.6(B:O) IC210.2(1A)
PROG_MODE: IC250.5(B:I1)
R_SHIFT_H_OUT: IC104.1(G1) IC104.19(G2)
R_SHIFT_H_WRT: IC82.1(G)
R_SHIFT_IN_SRC: IC94.1(!A!/B) IC95.1(!A!/B) IC96.1(!A!/B) IC97.1(!A!/B)
R_SHIFT_L_OUT: IC103.1(G1) IC103.19(G2)
R_SHIFT_L_WRT: IC93.1(G)
RD: IC69.9(B:Y1) R10.8
REQ_ENCOD_0: IC160.11(B:A1) IC222.1(A)
REQ_ENCOD_1: IC222.2(B) IC226.7(A1)
REQ_ENCOD_2: IC222.3(C) IC226.6(A2)
RST: IC54.3(B:I) IC128.15(CLR) IC139.15(CLR) IC144.15(CLR) IC248.15(CLR) IC249.15(CLR) R3.1 S2.2(P)
SF: IC46.6(3Q) IC59.11(3A) IC195.15(B:A3)
SF_FROM_ALU: IC126.7(3D)
SF_XOR_OF: IC72.6(B:O) IC81.4(B:I0) IC142.11(2C1)
SPH_OUT: IC111.19(B:G) IC112.19(B:G)
SPH_WRT: IC4.1(G)
SPL_OUT: IC109.19(B:G) IC110.19(B:G)
SPL_WRT: IC5.1(G)
STOP_CLK: IC44.2(A:D) IC44.5(A:Q) IC147.4(B:I0) R9.1 S4.2(P)
TDR0_H_WRT: IC239.1(G)
TDR0_H_X_OUT: IC237.1(A:G) IC238.1(A:G)
TDR0_L_WRT: IC240.1(G)
TDR0_L_X_OUT: IC235.8(A:A4)
TDR0H_WRT: IC17.1(G)
TDR0H_Y_OUT: IC213.1(A:G) IC214.1(A:G)
TDR0L_OUT3: IC229.1(A:G)
TDR0L_OUT4: IC235.1(A:G)
TDR0L_WRT: IC16.1(G)
TDR0L_Y_OUT: IC211.1(A:G) IC212.1(A:G)
TDR1_H_WRT: IC233.1(G)
TDR1_H_X_OUT: IC231.1(A:G) IC232.1(A:G)
TDR1_L_WRT: IC234.1(G)
TDR1_L_X_OUT: IC229.8(A:A4)
TDR1H_WRT: IC88.1(G)
TDR1H_Y_OUT: IC91.1(A:G) IC92.1(A:G)
TDR1L_WRT: IC86.1(G)
TDR1L_Y_OUT: IC89.1(A:G) IC90.1(A:G)
TRAP_IN: IC187.3(A:CLK) IC207.1(A:I0)
TYP_0: IC43.3(B:I) IC67.4(B:I0)
TYP_1: IC39.2(A:I1) IC42.1(A:I0) IC84.3(B:I)
U_AD0: IC32.2(Q1) IC140.2(A1) IC166.2(A1) U$6.10(A0) U$7.10(A0) U$8.10(A0) U$9.10(A0)
U_AD1: IC32.5(Q2) IC140.3(A2) IC166.3(A2) U$6.9(A1) U$7.9(A1) U$8.9(A1) U$9.9(A1)
U_AD2: IC32.6(Q3) IC140.4(A3) U$6.8(A2) U$7.8(A2) U$8.8(A2) U$9.8(A2)
U_AD3: IC32.9(Q4) IC140.5(A4) U$6.7(A3) U$7.7(A3) U$8.7(A3) U$9.7(A3)
U_AD4: IC32.12(Q5) IC140.6(A5) U$6.6(A4) U$7.6(A4) U$8.6(A4) U$9.6(A4)
U_AD5: IC32.15(Q6) IC140.7(A6) U$6.5(A5) U$7.5(A5) U$8.5(A5) U$9.5(A5)
U_AD6: IC32.16(Q7) IC140.8(A7) U$6.4(A6) U$7.4(A6) U$8.4(A6) U$9.4(A6)
U_AD7: IC32.19(Q8) IC140.9(A8) U$6.3(A7) U$7.3(A7) U$8.3(A7) U$9.3(A7)
U_AD8: IC33.2(Q1) U$6.25(A8) U$7.25(A8) U$8.25(A8) U$9.25(A8)
U_AD9: IC33.5(Q2) IC118.2(A1) IC118.3(A2) U$6.24(A9) U$7.24(A9) U$8.24(A9) U$9.24(A9)
U_AD10: IC33.6(Q3) IC118.4(A3) U$6.21(A10) U$7.21(A10) U$8.21(A10) U$9.21(A10)
U_AD11: IC33.9(Q4) IC118.5(A4) U$6.23(A11) U$7.23(A11) U$8.23(A11) U$9.23(A11)
U_AD12: IC33.12(Q5) IC118.6(A5) U$6.2(A12) U$7.2(A12) U$8.2(A12) U$9.2(A12)
U_AD13: IC33.15(Q6) IC118.7(A6) U$6.26(A13) U$7.26(A13) U$8.26(A13) U$9.26(A13)
U_AD_BUFF0: IC140.18(Y1) U$1.10(A0)
U_AD_BUFF1: IC140.17(Y2) U$1.9(A1)
U_AD_BUFF2: IC140.16(Y3) U$1.8(A2)
U_AD_BUFF3: IC140.15(Y4) U$1.7(A3)
U_AD_BUFF4: IC140.14(Y5) U$1.6(A4)
U_AD_BUFF5: IC140.13(Y6) U$1.5(A5)
U_AD_BUFF6: IC140.12(Y7) U$1.4(A6)
U_AD_BUFF7: IC140.11(Y8) U$1.3(A7)
U_AD_BUFF8: IC118.18(Y1) U$1.25(A8)
U_AD_BUFF9: IC118.17(Y2) U$1.24(A9)
U_AD_BUFF10: IC118.16(Y3) U$1.21(A10)
U_AD_BUFF11: IC118.15(Y4) U$1.23(A11)
U_AD_BUFF12: IC118.14(Y5) U$1.2(A12)
U_AD_BUFF13: IC118.13(Y6) U$1.26(A13)
U_ADDER_0: IC41.6(1C0) IC50.4(S1)
U_ADDER_1: IC41.10(2C0)
U_ADDER_2: IC40.6(1C0)
U_ADDER_3: IC40.10(2C0)
U_ADDER_4: IC34.6(1C0)
U_ADDER_5: IC34.10(2C0)
U_ADDER_6: IC35.6(1C0)
U_ADDER_7: IC35.10(2C0)
U_ADDER_8: IC36.6(1C0)
U_ADDER_9: IC36.10(2C0)
U_ADDER_10: IC37.6(1C0)
U_ADDER_11: IC37.10(2C0)
U_ADDER_12: IC38.6(1C0)
U_ADDER_13: IC38.10(2C0) IC53.1(S2)
U_ADDR_BUFF1_0: IC166.18(Y1)
U_ADDR_BUFF1_1: IC166.17(Y2)
U_ADDR_BUFF1_13: IC165.13(Y6)
U_ADDR_MUX_0: IC34.14(A) IC35.14(A) IC36.14(A) IC37.14(A) IC38.14(A) IC39.3(A:O) IC40.14(A) IC41.14(A)
U_ADDR_MUX_1: IC34.2(B) IC35.2(B) IC36.2(B) IC37.2(B) IC38.2(B) IC40.2(B) IC41.2(B) IC42.3(A:O)
U_CF: IC59.6(2B) IC126.5(2Q) IC167.3(1B)
U_DMA_ADDR_0: IC173.3(1B)
U_DMA_ADDR_1: IC173.6(2B)
U_DMA_ADDR_2: IC173.10(3B)
U_DMA_ADDR_3: IC173.13(4B)
U_DMA_ADDR_4: IC169.3(1B)
U_DMA_ADDR_5: IC169.6(2B)
U_DMA_ADDR_6: IC169.10(3B)
U_DMA_ADDR_7: IC169.13(4B)
U_DMA_ADDR_8: IC171.3(1B)
U_DMA_ADDR_9: IC171.6(2B)
U_DMA_ADDR_10: IC171.10(3B)
U_DMA_ADDR_11: IC171.13(4B)
U_DMA_ADDR_12: IC172.3(1B)
U_DMA_ADDR_13: IC172.6(2B)
U_FETCH_0: IC41.5(1C1) R7.16 SW1.1
U_FETCH_1: IC41.11(2C1)
U_FETCH_2: IC40.5(1C1)
U_FETCH_3: IC40.11(2C1)
U_FETCH_4: IC34.5(1C1)
U_FETCH_5: IC34.11(2C1)
U_FETCH_6: IC35.5(1C1)
U_FETCH_7: IC35.11(2C1)
U_FETCH_8: IC36.5(1C1)
U_FETCH_9: IC36.11(2C1)
U_FETCH_10: IC37.5(1C1)
U_FETCH_11: IC37.11(2C1)
U_FETCH_12: IC38.5(1C1)
U_FETCH_13: IC38.11(2C1) R6.1 SW2.8
U_FLAGS_REG_WRT: IC126.1(G)
U_INT_ADDR_0: IC173.2(1A)
U_INT_ADDR_1: IC173.5(2A)
U_INT_ADDR_2: IC173.11(3A)
U_INT_ADDR_3: IC173.14(4A)
U_INT_ADDR_4: IC169.2(1A)
U_INT_ADDR_5: IC169.5(2A)
U_INT_ADDR_6: IC169.11(3A)
U_INT_ADDR_7: IC169.14(4A)
U_INT_ADDR_8: IC171.2(1A)
U_INT_ADDR_9: IC171.5(2A)
U_INT_ADDR_10: IC171.11(3A)
U_INT_ADDR_11: IC171.14(4A)
U_INT_ADDR_12: IC172.2(1A)
U_INT_ADDR_13: IC172.5(2A)
U_OF: IC59.13(4B) IC126.9(4Q)
U_REQ_ADDR_0: IC41.3(1C3) IC173.4(1Y)
U_REQ_ADDR_1: IC41.13(2C3) IC173.7(2Y)
U_REQ_ADDR_2: IC40.3(1C3) IC173.9(3Y)
U_REQ_ADDR_3: IC40.13(2C3) IC173.12(4Y)
U_REQ_ADDR_4: IC34.3(1C3) IC169.4(1Y)
U_REQ_ADDR_5: IC34.13(2C3) IC169.7(2Y)
U_REQ_ADDR_6: IC35.3(1C3) IC169.9(3Y)
U_REQ_ADDR_7: IC35.13(2C3) IC169.12(4Y)
U_REQ_ADDR_8: IC36.3(1C3) IC171.4(1Y)
U_REQ_ADDR_9: IC36.13(2C3) IC171.7(2Y)
U_REQ_ADDR_10: IC37.3(1C3) IC171.9(3Y)
U_REQ_ADDR_11: IC37.13(2C3) IC171.12(4Y)
U_REQ_ADDR_12: IC38.3(1C3) IC172.4(1Y)
U_REQ_ADDR_13: IC38.13(2C3) IC172.7(2Y)
U_SF: IC59.10(3B) IC126.6(3Q)
U_ZF: IC59.3(1B) IC126.2(1Q) IC127.2(A:I1)
U_ZF_IN_SRC: IC121.1(!A!/B)
VCC: IC44.1(A:CLR) IC49.2(1A) IC56.5(1C1) IC163.2(A:D) IC163.4(A:PRE) IC164.2(A:D) IC164.4(A:PRE) IC168.2(A:D) IC168.4(A:PRE) IC174.2(A:D) IC174.4(A:PRE) IC187.2(A:D) IC187.4(A:PRE) IC188.2(A:D) IC188.4(A:PRE) IC221.2(A:D) IC221.4(A:PRE) IC222.6(G1) R1.2 R2.2 R3.2 R9.2 SW1.9 SW1.10 SW1.11 SW1.12 SW1.13 SW1.14 SW1.15 SW1.16 SW2.9 SW2.10 SW2.11 SW2.12 SW2.13 SW2.14 SW2.15 SW2.16
WR: IC69.7(B:Y2) R10.7
XBUS0: IC2.9(B:Y1) IC8.9(B:Y1) IC9.18(A:Y1) IC25.9(B:Y1) IC27.9(B:Y1) IC102.9(B:Y1) IC103.18(Y1) IC104.18(Y1) IC105.9(B:Y1) IC107.9(B:Y1) IC109.9(B:Y1) IC111.9(B:Y1) IC113.9(B:Y1) IC115.9(B:Y1) IC145.9(B:Y1) IC156.9(B:Y1) IC160.9(B:Y1) IC181.18(A:Y1) IC186.9(B:Y1) IC195.9(B:Y1) IC244.9(B:Y1) R8.9
XBUS1: IC2.7(B:Y2) IC8.7(B:Y2) IC9.16(A:Y2) IC25.7(B:Y2) IC27.7(B:Y2) IC102.7(B:Y2) IC104.17(Y2) IC105.7(B:Y2) IC107.7(B:Y2) IC109.7(B:Y2) IC111.7(B:Y2) IC113.7(B:Y2) IC115.7(B:Y2) IC145.7(B:Y2) IC156.7(B:Y2) IC160.7(B:Y2) IC181.16(A:Y2) IC186.7(B:Y2) IC195.7(B:Y2) IC244.7(B:Y2) R8.10
XBUS2: IC2.5(B:Y3) IC8.5(B:Y3) IC9.14(A:Y3) IC25.5(B:Y3) IC27.5(B:Y3) IC102.5(B:Y3) IC105.5(B:Y3) IC107.5(B:Y3) IC109.5(B:Y3) IC111.5(B:Y3) IC113.5(B:Y3) IC115.5(B:Y3) IC145.5(B:Y3) IC156.5(B:Y3) IC160.5(B:Y3) IC181.14(A:Y3) IC186.5(B:Y3) IC195.5(B:Y3) IC244.5(B:Y3) R8.11
XBUS3: IC2.3(B:Y4) IC8.3(B:Y4) IC9.12(A:Y4) IC25.3(B:Y4) IC27.3(B:Y4) IC102.3(B:Y4) IC105.3(B:Y4) IC107.3(B:Y4) IC109.3(B:Y4) IC111.3(B:Y4) IC113.3(B:Y4) IC115.3(B:Y4) IC145.3(B:Y4) IC156.3(B:Y4) IC160.3(B:Y4) IC181.12(A:Y4) IC186.3(B:Y4) IC195.3(B:Y4) IC244.3(B:Y4) R8.12
XBUS4: IC3.9(B:Y1) IC9.9(B:Y1) IC24.9(B:Y1) IC26.9(B:Y1) IC103.14(Y5) IC106.9(B:Y1) IC108.9(B:Y1) IC110.9(B:Y1) IC112.9(B:Y1) IC114.9(B:Y1) IC116.9(B:Y1) IC117.9(B:Y1) IC129.9(B:Y1) IC146.9(B:Y1) IC159.9(B:Y1) IC161.9(B:Y1) IC176.18(A:Y1) IC196.9(B:Y1) IC215.9(B:Y1) IC247.9(B:Y1) R8.13
XBUS5: IC3.7(B:Y2) IC9.7(B:Y2) IC24.7(B:Y2) IC26.7(B:Y2) IC106.7(B:Y2) IC108.7(B:Y2) IC110.7(B:Y2) IC112.7(B:Y2) IC114.7(B:Y2) IC116.7(B:Y2) IC117.7(B:Y2) IC129.7(B:Y2) IC146.7(B:Y2) IC159.7(B:Y2) IC161.7(B:Y2) IC176.16(A:Y2) IC196.7(B:Y2) IC215.7(B:Y2) IC247.7(B:Y2) R8.14
XBUS6: IC3.5(B:Y3) IC9.5(B:Y3) IC24.5(B:Y3) IC26.5(B:Y3) IC106.5(B:Y3) IC108.5(B:Y3) IC110.5(B:Y3) IC112.5(B:Y3) IC114.5(B:Y3) IC116.5(B:Y3) IC117.5(B:Y3) IC129.5(B:Y3) IC146.5(B:Y3) IC159.5(B:Y3) IC161.5(B:Y3) IC176.14(A:Y3) IC196.5(B:Y3) IC215.5(B:Y3) IC247.5(B:Y3) R8.15
XBUS7: IC3.3(B:Y4) IC9.3(B:Y4) IC24.3(B:Y4) IC26.3(B:Y4) IC80.4(B:I0) IC103.11(Y8) IC104.11(Y8) IC106.3(B:Y4) IC108.3(B:Y4) IC110.3(B:Y4) IC112.3(B:Y4) IC114.3(B:Y4) IC116.3(B:Y4) IC117.3(B:Y4) IC129.3(B:Y4) IC130.5(B:I1) IC146.3(B:Y4) IC159.3(B:Y4) IC161.3(B:Y4) IC176.12(A:Y4) IC196.3(B:Y4) IC215.3(B:Y4) IC247.3(B:Y4) R8.16
XBUS8: IC154.9(B:Y1)
XBUS9: IC154.7(B:Y2)
XBUS10: IC154.5(B:Y3)
XBUS11: IC154.3(B:Y4)
XBUS12: IC155.9(B:Y1)
XBUS13: IC155.7(B:Y2)
XBUS14: IC155.5(B:Y3)
XBUS15: IC155.3(B:Y4)
XBUS16: IC89.18(A:Y1) IC91.18(A:Y1)
XBUS17: IC89.16(A:Y2) IC91.16(A:Y2)
XBUS18: IC89.14(A:Y3) IC91.14(A:Y3)
XBUS19: IC89.12(A:Y4) IC91.12(A:Y4)
XBUS20: IC90.18(A:Y1) IC92.18(A:Y1)
XBUS21: IC90.16(A:Y2) IC92.16(A:Y2)
XBUS22: IC90.14(A:Y3) IC92.14(A:Y3)
XBUS23: IC90.12(A:Y4) IC92.12(A:Y4)
XBUS32: IC122.18(A:Y1)
XBUS33: IC122.16(A:Y2)
XBUS34: IC122.14(A:Y3)
XBUS35: IC122.12(A:Y4)
XBUS36: IC122.9(B:Y1)
XBUS37: IC122.7(B:Y2)
XBUS38: IC122.5(B:Y3)
XBUS39: IC122.3(B:Y4)
XBUS40: IC124.9(B:Y1)
XBUS41: IC124.7(B:Y2)
XBUS42: IC124.5(B:Y3)
XBUS43: IC124.3(B:Y4)
XBUS44: IC125.9(B:Y1)
XBUS45: IC125.7(B:Y2)
XBUS46: IC125.5(B:Y3)
XBUS47: IC125.3(B:Y4)
XBUS48: IC217.18(A:Y1)
XBUS49: IC217.16(A:Y2)
XBUS50: IC217.14(A:Y3)
XBUS51: IC217.12(A:Y4)
XBUS52: IC217.9(B:Y1)
XBUS53: IC217.7(B:Y2)
XBUS54: IC217.5(B:Y3)
XBUS55: IC217.3(B:Y4)
YBUS0: IC19.18(A:Y1) IC182.18(A:Y1)
YBUS1: IC19.16(A:Y2) IC182.16(A:Y2)
YBUS2: IC19.14(A:Y3) IC182.14(A:Y3)
YBUS3: IC19.12(A:Y4) IC182.12(A:Y4)
YBUS4: IC19.9(B:Y1) IC183.18(A:Y1)
YBUS5: IC19.7(B:Y2) IC183.16(A:Y2)
YBUS6: IC19.5(B:Y3) IC183.14(A:Y3)
YBUS7: IC19.3(B:Y4) IC130.4(B:I0) IC183.12(A:Y4)
YBUS16: IC211.18(A:Y1) IC213.18(A:Y1)
YBUS17: IC211.16(A:Y2) IC213.16(A:Y2)
YBUS18: IC211.14(A:Y3) IC213.14(A:Y3)
YBUS19: IC211.12(A:Y4) IC213.12(A:Y4)
YBUS20: IC212.18(A:Y1) IC214.18(A:Y1)
YBUS21: IC212.16(A:Y2) IC214.16(A:Y2)
YBUS22: IC212.14(A:Y3) IC214.14(A:Y3)
YBUS23: IC212.12(A:Y4) IC214.12(A:Y4)
YBUS40: IC229.18(A:Y1) IC231.18(A:Y1)
YBUS41: IC229.16(A:Y2) IC231.16(A:Y2)
YBUS42: IC229.14(A:Y3) IC231.14(A:Y3)
YBUS43: IC229.12(A:Y4) IC231.12(A:Y4)
YBUS44: IC230.18(A:Y1) IC232.18(A:Y1)
YBUS45: IC230.16(A:Y2) IC232.16(A:Y2)
YBUS46: IC230.14(A:Y3) IC232.14(A:Y3)
YBUS47: IC230.12(A:Y4) IC232.12(A:Y4)
YBUS48: IC235.18(A:Y1) IC237.18(A:Y1)
YBUS49: IC235.16(A:Y2) IC237.16(A:Y2)
YBUS50: IC235.14(A:Y3) IC237.14(A:Y3)
YBUS51: IC235.12(A:Y4) IC237.12(A:Y4)
YBUS52: IC236.18(A:Y1) IC238.18(A:Y1)
YBUS53: IC236.16(A:Y2) IC238.16(A:Y2)
YBUS54: IC236.14(A:Y3) IC238.14(A:Y3)
YBUS55: IC236.12(A:Y4) IC238.12(A:Y4)
ZBUFF0_16: IC86.3(1D) IC88.3(1D)
ZBUFF0_17: IC86.4(2D) IC88.4(2D)
ZBUFF0_18: IC86.7(3D) IC88.7(3D)
ZBUFF0_19: IC86.8(4D) IC88.8(4D)
ZBUFF0_20: IC86.13(5D) IC88.13(5D)
ZBUFF0_21: IC88.14(6D)
ZBUFF0_22: IC86.14(6D) IC86.17(7D) IC88.17(7D)
ZBUFF0_23: IC86.18(8D) IC88.18(8D)
ZBUFF0_24: IC16.3(1D) IC17.3(1D)
ZBUFF0_25: IC16.4(2D) IC17.4(2D)
ZBUFF0_26: IC16.7(3D) IC17.7(3D)
ZBUFF0_27: IC16.8(4D) IC17.8(4D)
ZBUFF0_28: IC16.13(5D) IC17.13(5D)
ZBUFF0_29: IC16.14(6D) IC17.14(6D)
ZBUFF0_30: IC16.17(7D) IC17.17(7D)
ZBUFF0_31: IC16.18(8D) IC17.18(8D)
ZBUFF0_56: IC233.3(1D) IC234.3(1D)
ZBUFF0_57: IC233.4(2D) IC234.4(2D)
ZBUFF0_58: IC233.7(3D) IC234.7(3D)
ZBUFF0_59: IC233.8(4D) IC234.8(4D)
ZBUFF0_60: IC233.13(5D) IC234.13(5D)
ZBUFF0_61: IC233.14(6D) IC234.14(6D)
ZBUFF0_62: IC233.17(7D) IC234.17(7D)
ZBUFF0_63: IC233.18(8D) IC234.18(8D)
ZBUFF0_64: IC239.3(1D) IC240.3(1D)
ZBUFF0_65: IC239.4(2D) IC240.4(2D)
ZBUFF0_66: IC239.7(3D) IC240.7(3D)
ZBUFF0_67: IC239.8(4D) IC240.8(4D)
ZBUFF0_68: IC239.13(5D) IC240.13(5D)
ZBUFF0_69: IC239.14(6D) IC240.14(6D)
ZBUFF0_70: IC239.17(7D) IC240.17(7D)
ZBUFF0_71: IC239.18(8D) IC240.18(8D)
ZBUFF1_0: IC4.3(1D) IC5.3(1D) IC98.3(1D) IC99.3(1D)
ZBUFF1_1: IC4.4(2D) IC5.4(2D) IC98.4(2D) IC99.4(2D)
ZBUFF1_2: IC4.7(3D) IC5.7(3D) IC98.7(3D) IC99.7(3D)
ZBUFF1_3: IC4.8(4D) IC5.8(4D) IC98.8(4D) IC99.8(4D)
ZBUFF1_4: IC4.13(5D) IC5.13(5D) IC98.13(5D) IC99.13(5D)
ZBUFF1_5: IC4.14(6D) IC5.14(6D) IC98.14(6D) IC99.14(6D)
ZBUFF1_6: IC4.17(7D) IC5.17(7D) IC98.17(7D) IC99.17(7D)
ZBUFF1_7: IC4.18(8D) IC5.18(8D) IC98.18(8D) IC99.18(8D)
ZBUFF2_0: IC1.3(1D) IC23.14(4A) IC100.3(1D) IC101.3(1D)
ZBUFF2_1: IC1.4(2D) IC23.11(3A) IC100.4(2D) IC101.4(2D)
ZBUFF2_2: IC1.7(3D) IC23.5(2A) IC100.7(3D) IC101.7(3D)
ZBUFF2_3: IC1.8(4D) IC23.2(1A) IC100.8(4D) IC101.8(4D)
ZBUFF2_4: IC1.13(5D) IC22.14(4A) IC100.13(5D) IC101.13(5D)
ZBUFF2_5: IC1.14(6D) IC22.11(3A) IC100.14(6D) IC101.14(6D)
ZBUFF2_6: IC1.17(7D) IC22.5(2A) IC100.17(7D) IC101.17(7D)
ZBUFF2_7: IC22.2(1A) IC100.18(8D) IC101.18(8D)
ZBUFF2_16: IC123.3(1D)
ZBUFF2_17: IC123.4(2D)
ZBUFF2_18: IC123.7(3D)
ZBUFF2_19: IC123.8(4D)
ZBUFF2_20: IC123.13(5D)
ZBUFF2_21: IC123.14(6D)
ZBUFF2_22: IC123.17(7D)
ZBUFF2_23: IC153.3(1D)
ZBUFF2_24: IC153.4(2D)
ZBUFF2_25: IC153.7(3D)
ZBUFF2_26: IC153.8(4D)
ZBUFF2_27: IC153.13(5D)
ZBUFF2_28: IC153.14(6D)
ZBUFF2_29: IC153.17(7D)
ZBUFF2_30: IC153.18(8D)
ZBUFF2_31: IC185.3(1D)
ZBUFF2_32: IC185.4(2D)
ZBUFF2_33: IC185.7(3D)
ZBUFF2_34: IC185.8(4D)
ZBUFF2_35: IC185.13(5D)
ZBUFF2_36: IC185.14(6D)
ZBUFF2_37: IC185.17(7D)
ZBUFF2_38: IC185.18(8D)
ZBUS0: IC6.3(1D) IC7.3(1D) IC47.3(1B) IC48.3(1D) IC96.2(1A) IC97.2(1A) IC144.14(D1) IC175.4(B:I0) IC184.3(1D) IC189.3(1D) IC197.1(A:I0) IC216.3(1D) IC245.18(A:Y1) IC248.14(D1)
ZBUS1: IC14.10(F1) IC47.6(2B) IC96.5(2A) IC97.5(2A) IC144.13(D2) IC175.5(B:I1) IC184.4(2D) IC197.2(A:I1) IC216.4(2D) IC245.4(A:A2) IC245.16(A:Y2) IC248.13(D2)
ZBUS2: IC14.11(F2) IC47.10(3B) IC96.11(3A) IC97.11(3A) IC144.12(D3) IC177.5(B:I1) IC184.7(3D) IC197.3(A:I2) IC216.7(3D) IC245.6(A:A3) IC245.14(A:Y3) IC248.12(D3)
ZBUS3: IC14.13(F3) IC47.13(4B) IC96.14(4A) IC97.14(4A) IC144.11(D4) IC184.8(4D) IC192.5(B:I1) IC197.12(A:I3) IC216.8(4D) IC245.8(A:A4) IC245.12(A:Y4) IC248.11(D4)
ZBUS4: IC15.13(F3) IC94.2(1A) IC95.2(1A) IC128.14(D1) IC184.13(5D) IC193.5(B:I1) IC197.13(A:I4) IC210.3(1B) IC216.13(5D) IC246.8(A:A4) IC246.18(A:Y1) IC249.14(D1)
ZBUS5: IC15.11(F2) IC94.5(2A) IC95.5(2A) IC128.13(D2) IC184.14(6D) IC194.5(B:I1) IC199.2(A:I1) IC216.14(6D) IC246.6(A:A3) IC246.16(A:Y2) IC249.13(D2)
ZBUS6: IC15.10(F1) IC94.11(3A) IC95.11(3A) IC128.12(D3) IC184.17(7D) IC199.3(A:I2) IC200.5(B:I1) IC216.17(7D) IC246.4(A:A2) IC246.14(A:Y3) IC249.12(D3)
ZBUS7: IC6.18(8D) IC7.18(8D) IC15.9(F0) IC47.11(3A) IC48.18(8D) IC80.5(B:I1) IC94.14(4A) IC95.14(4A) IC128.11(D4) IC184.18(8D) IC189.18(8D) IC199.12(A:I3) IC209.5(B:I1) IC216.18(8D) IC246.2(A:A1) IC246.12(A:Y4) IC249.11(D4)
ZF: IC46.2(1Q) IC59.2(1A) IC120.2(A:I1) IC195.11(B:A1)
ZF_FROM_ALU: IC119.2(1A) IC120.1(A:I0) IC121.2(1A) IC127.1(A:I0) IC199.5(A:O)
ZF_IN_SRC: IC119.1(!A!/B)
~RST: IC44.4(A:PRE) IC54.4(B:O) IC162.1(CLR) IC208.1(A:I0) IC218.1(A:I0) IC219.1(A:I0) IC220.2(A:I1) IC223.2(A:I1) IC224.2(A:I1) IC225.2(A:I1)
